FUNCTION "Gest Aut Robot Boxing DX" : VOID
TITLE =Gestione Ciclo Automatico Robot 3 Piantaggi
AUTHOR : MassimoZ
FAMILY : NovaSrl
VERSION : 0.1

BEGIN
NETWORK
TITLE ======== CICLO BOXING DX ======



NETWORK
TITLE ======== Primo Prelievo Ciclo 3 Pinataggi Boxing =======



NETWORK
TITLE =Com Aut Start Primo Posizionamento di Prelievo Asse X Boxing DX
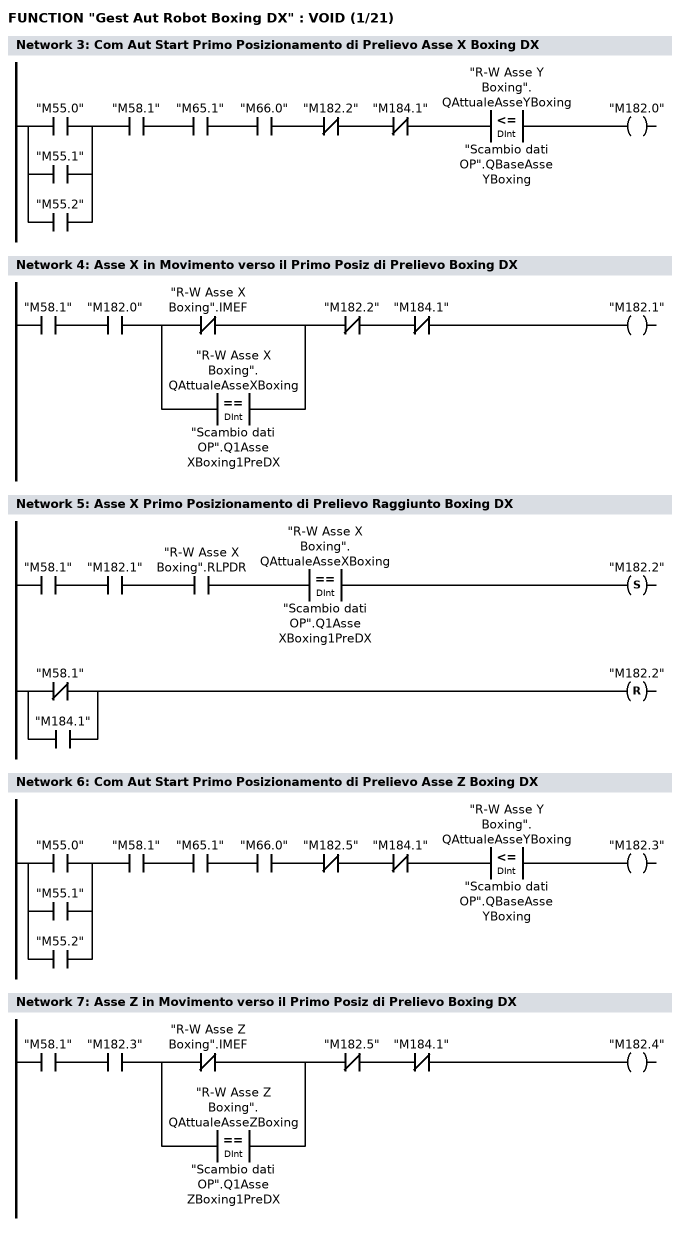
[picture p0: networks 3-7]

      U(    ;
      O     "M55.0";
      O     "M55.1";
      O     "M55.2";
      )     ;
      U     "M58.1";
      U     "M65.1";
      U     "M66.0";
      UN    "M182.2";
      UN    "M184.1";
      U(    ;
      L     "R-W Asse Y Boxing".QAttualeAsseYBoxing;
      L     "Scambio dati OP".QBaseAsseYBoxing;
      <=D   ;
      )     ;
      =     "M182.0";
NETWORK
TITLE =Asse X in Movimento verso il Primo Posiz di Prelievo Boxing DX

      U     "M58.1";
      U     "M182.0";
      U(    ;
      ON    "R-W Asse X Boxing".IMEF;
      O(    ;
      L     "R-W Asse X Boxing".QAttualeAsseXBoxing;
      L     "Scambio dati OP".Q1AsseXBoxing1PreDX;
      ==D   ;
      )     ;
      )     ;
      UN    "M182.2";
      UN    "M184.1";
      =     "M182.1";
NETWORK
TITLE =Asse X Primo Posizionamento di Prelievo Raggiunto Boxing DX

      U     "M58.1";
      U     "M182.1";
      U     "R-W Asse X Boxing".RLPDR;
      U(    ;
      L     "R-W Asse X Boxing".QAttualeAsseXBoxing;
      L     "Scambio dati OP".Q1AsseXBoxing1PreDX;
      ==D   ;
      )     ;
      S     "M182.2";
      U(    ;
      ON    "M58.1";
      O     "M184.1";
      )     ;
      R     "M182.2";
      NOP   0;
NETWORK
TITLE =Com Aut Start Primo Posizionamento di Prelievo Asse Z Boxing DX

      U(    ;
      O     "M55.0";
      O     "M55.1";
      O     "M55.2";
      )     ;
      U     "M58.1";
      U     "M65.1";
      U     "M66.0";
      UN    "M182.5";
      UN    "M184.1";
      U(    ;
      L     "R-W Asse Y Boxing".QAttualeAsseYBoxing;
      L     "Scambio dati OP".QBaseAsseYBoxing;
      <=D   ;
      )     ;
      =     "M182.3";
NETWORK
TITLE =Asse Z in Movimento verso il Primo Posiz di Prelievo Boxing DX

      U     "M58.1";
      U     "M182.3";
      U(    ;
      ON    "R-W Asse Z Boxing".IMEF;
      O(    ;
      L     "R-W Asse Z Boxing".QAttualeAsseZBoxing;
      L     "Scambio dati OP".Q1AsseZBoxing1PreDX;
      ==D   ;
      )     ;
      )     ;
      UN    "M182.5";
      UN    "M184.1";
      =     "M182.4";
NETWORK
TITLE =Asse Z Primo Posizionamento di Prelievo Raggiunto Boxing DX
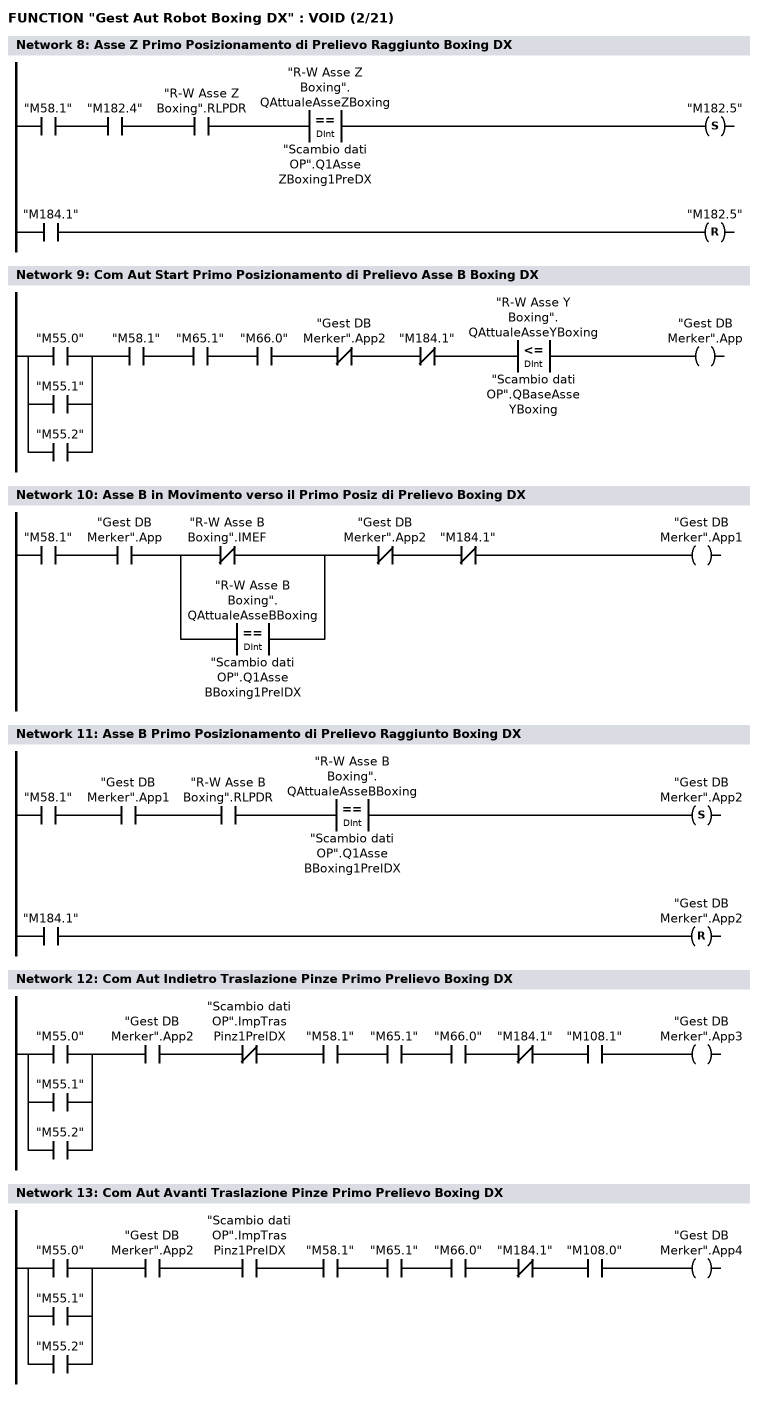
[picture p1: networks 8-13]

      U     "M58.1";
      U     "M182.4";
      U     "R-W Asse Z Boxing".RLPDR;
      U(    ;
      L     "R-W Asse Z Boxing".QAttualeAsseZBoxing;
      L     "Scambio dati OP".Q1AsseZBoxing1PreDX;
      ==D   ;
      )     ;
      S     "M182.5";
      U     "M184.1";
      R     "M182.5";
      NOP   0;
NETWORK
TITLE =Com Aut Start Primo Posizionamento di Prelievo Asse B Boxing DX



      U(    ;
      O     "M55.0";
      O     "M55.1";
      O     "M55.2";
      )     ;
      U     "M58.1";
      U     "M65.1";
      U     "M66.0";
      UN    "Gest DB Merker".App2;
      UN    "M184.1";
      U(    ;
      L     "R-W Asse Y Boxing".QAttualeAsseYBoxing;
      L     "Scambio dati OP".QBaseAsseYBoxing;
      <=D   ;
      )     ;
      =     "Gest DB Merker".App;
NETWORK
TITLE =Asse B in Movimento verso il Primo Posiz di Prelievo Boxing DX

      U     "M58.1";
      U     "Gest DB Merker".App;
      U(    ;
      ON    "R-W Asse B Boxing".IMEF;
      O(    ;
      L     "R-W Asse B Boxing".QAttualeAsseBBoxing;
      L     "Scambio dati OP".Q1AsseBBoxing1PrelDX;
      ==D   ;
      )     ;
      )     ;
      UN    "Gest DB Merker".App2;
      UN    "M184.1";
      =     "Gest DB Merker".App1;
NETWORK
TITLE =Asse B Primo Posizionamento di Prelievo Raggiunto Boxing DX

      U     "M58.1";
      U     "Gest DB Merker".App1;
      U     "R-W Asse B Boxing".RLPDR;
      U(    ;
      L     "R-W Asse B Boxing".QAttualeAsseBBoxing;
      L     "Scambio dati OP".Q1AsseBBoxing1PrelDX;
      ==D   ;
      )     ;
      S     "Gest DB Merker".App2;
      U     "M184.1";
      R     "Gest DB Merker".App2;
      NOP   0;
NETWORK
TITLE =Com Aut Indietro Traslazione Pinze Primo Prelievo Boxing DX

      U(    ;
      O     "M55.0";
      O     "M55.1";
      O     "M55.2";
      )     ;
      U     "Gest DB Merker".App2;
      UN    "Scambio dati OP".ImpTrasPinz1PrelDX;
      U     "M58.1";
      U     "M65.1";
      U     "M66.0";
      UN    "M184.1";
      U     "M108.1";
      =     "Gest DB Merker".App3;
NETWORK
TITLE =Com Aut Avanti Traslazione Pinze Primo Prelievo Boxing DX

      U(    ;
      O     "M55.0";
      O     "M55.1";
      O     "M55.2";
      )     ;
      U     "Gest DB Merker".App2;
      U     "Scambio dati OP".ImpTrasPinz1PrelDX;
      U     "M58.1";
      U     "M65.1";
      U     "M66.0";
      UN    "M184.1";
      U     "M108.0";
      =     "Gest DB Merker".App4;
NETWORK
TITLE =Com Aut Apertura Pinze Primo Prelievo Boxing DX
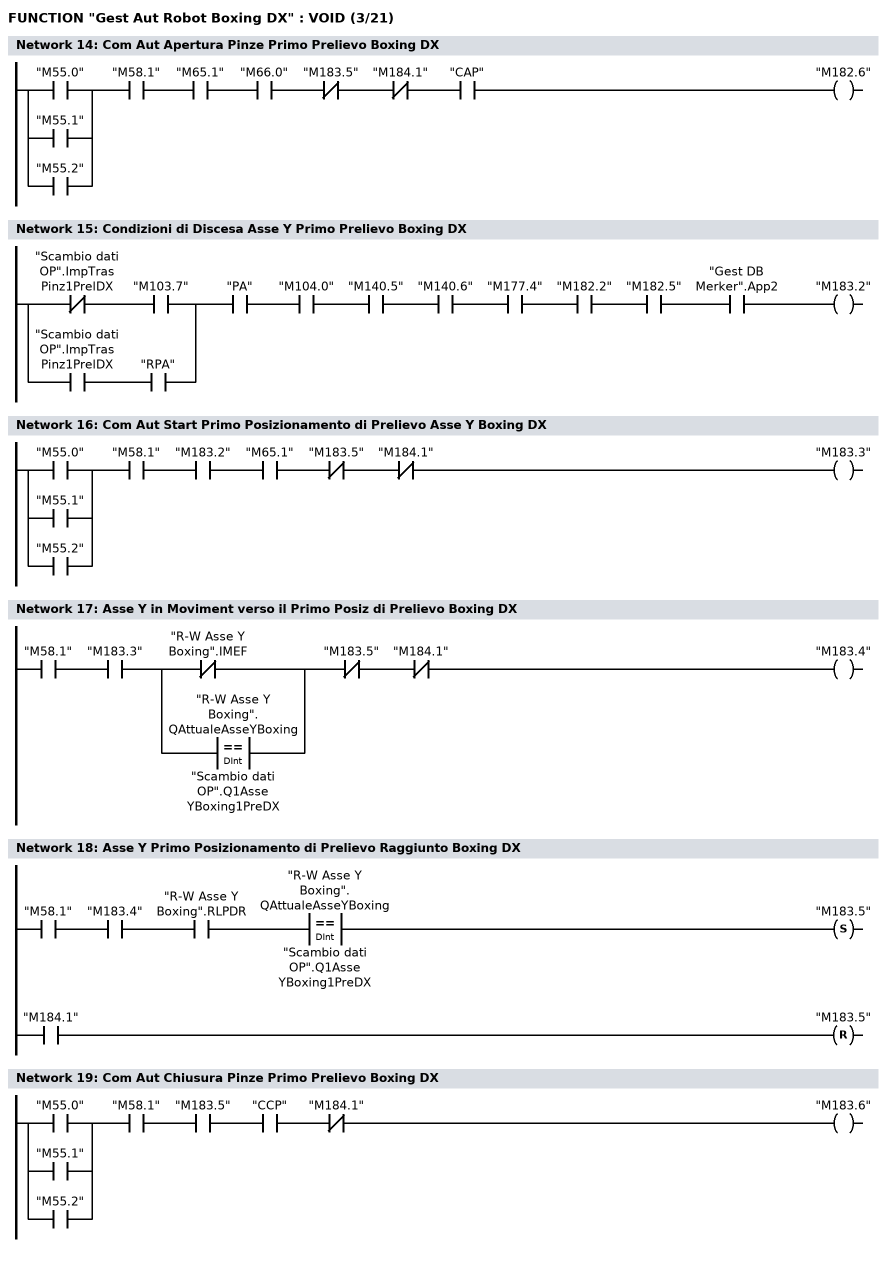
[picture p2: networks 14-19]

      U(    ;
      O     "M55.0";
      O     "M55.1";
      O     "M55.2";
      )     ;
      U     "M58.1";
      U     "M65.1";
      U     "M66.0";
      UN    "M183.5";
      UN    "M184.1";
      U     "CAP";
      =     "M182.6";
NETWORK
TITLE =Condizioni di Discesa Asse Y Primo Prelievo Boxing DX

      U(    ;
      UN    "Scambio dati OP".ImpTrasPinz1PrelDX;
      U     "M103.7";
      O     ;
      U     "Scambio dati OP".ImpTrasPinz1PrelDX;
      U     "RPA";
      )     ;
      U     "PA";
      U     "M104.0";
      U     "M140.5";
      U     "M140.6";
      U     "M177.4";
      U     "M182.2";
      U     "M182.5";
      U     "Gest DB Merker".App2;
      =     "M183.2";
NETWORK
TITLE =Com Aut Start Primo Posizionamento di Prelievo Asse Y Boxing DX

      U(    ;
      O     "M55.0";
      O     "M55.1";
      O     "M55.2";
      )     ;
      U     "M58.1";
      U     "M183.2";
      U     "M65.1";
      UN    "M183.5";
      UN    "M184.1";
      =     "M183.3";
NETWORK
TITLE =Asse Y in Moviment verso il Primo Posiz di Prelievo Boxing DX

      U     "M58.1";
      U     "M183.3";
      U(    ;
      ON    "R-W Asse Y Boxing".IMEF;
      O(    ;
      L     "R-W Asse Y Boxing".QAttualeAsseYBoxing;
      L     "Scambio dati OP".Q1AsseYBoxing1PreDX;
      ==D   ;
      )     ;
      )     ;
      UN    "M183.5";
      UN    "M184.1";
      =     "M183.4";
NETWORK
TITLE =Asse Y Primo Posizionamento di Prelievo Raggiunto Boxing DX

      U     "M58.1";
      U     "M183.4";
      U     "R-W Asse Y Boxing".RLPDR;
      U(    ;
      L     "R-W Asse Y Boxing".QAttualeAsseYBoxing;
      L     "Scambio dati OP".Q1AsseYBoxing1PreDX;
      ==D   ;
      )     ;
      S     "M183.5";
      U     "M184.1";
      R     "M183.5";
      NOP   0;
NETWORK
TITLE =Com Aut Chiusura Pinze Primo Prelievo Boxing DX

      U(    ;
      O     "M55.0";
      O     "M55.1";
      O     "M55.2";
      )     ;
      U     "M58.1";
      U     "M183.5";
      U     "CCP";
      UN    "M184.1";
      =     "M183.6";
NETWORK
TITLE =Tempo Chiusura Pinze Primo Prelievo Boxing DX
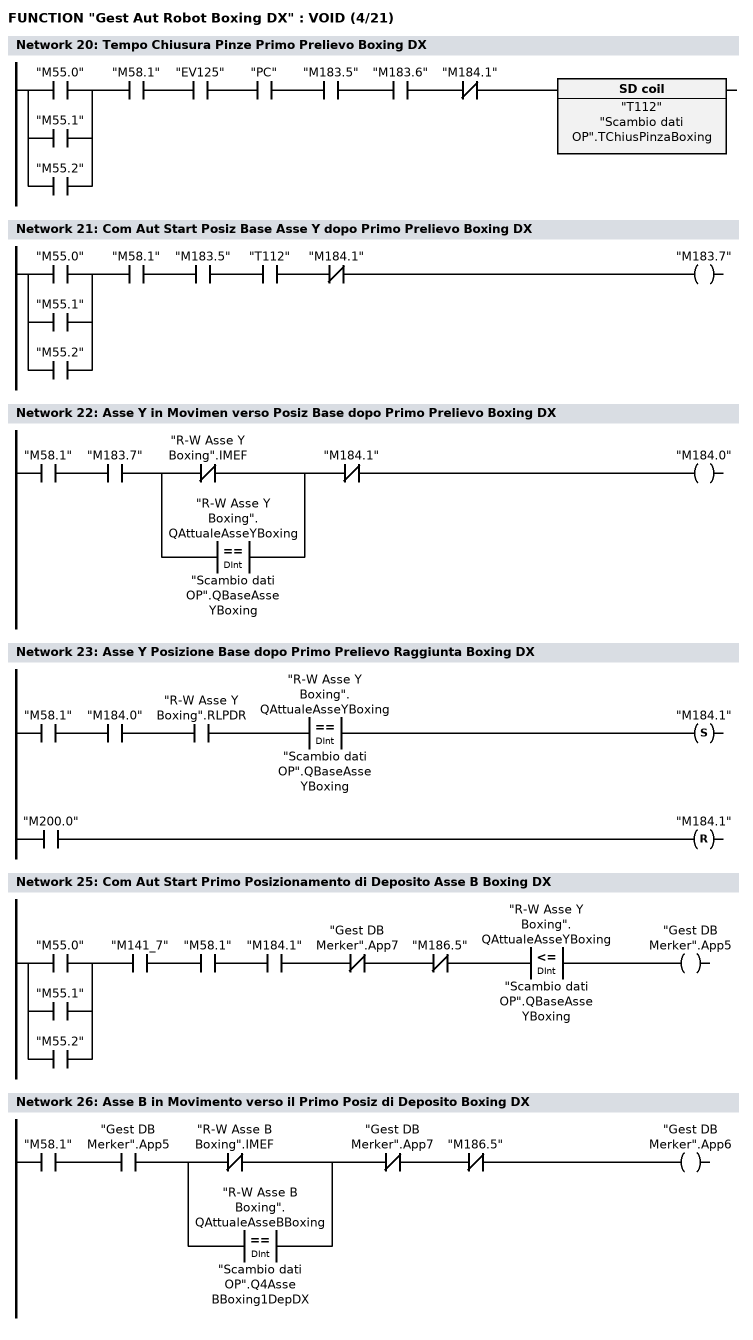
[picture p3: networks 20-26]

      U(    ;
      O     "M55.0";
      O     "M55.1";
      O     "M55.2";
      )     ;
      U     "M58.1";
      U     "EV125";
      U     "PC";
      U     "M183.5";
      U     "M183.6";
      UN    "M184.1";
      L     "Scambio dati OP".TChiusPinzaBoxing;
      SE    "T112";
      NOP   0;
      NOP   0;
      NOP   0;
      NOP   0;
NETWORK
TITLE =Com Aut Start Posiz Base Asse Y dopo Primo Prelievo Boxing DX

      U(    ;
      O     "M55.0";
      O     "M55.1";
      O     "M55.2";
      )     ;
      U     "M58.1";
      U     "M183.5";
      U     "T112";
      UN    "M184.1";
      =     "M183.7";
NETWORK
TITLE =Asse Y in Movimen verso Posiz Base dopo Primo Prelievo Boxing DX

      U     "M58.1";
      U     "M183.7";
      U(    ;
      ON    "R-W Asse Y Boxing".IMEF;
      O(    ;
      L     "R-W Asse Y Boxing".QAttualeAsseYBoxing;
      L     "Scambio dati OP".QBaseAsseYBoxing;
      ==D   ;
      )     ;
      )     ;
      UN    "M184.1";
      =     "M184.0";
NETWORK
TITLE =Asse Y Posizione Base dopo Primo Prelievo Raggiunta Boxing DX

      U     "M58.1";
      U     "M184.0";
      U     "R-W Asse Y Boxing".RLPDR;
      U(    ;
      L     "R-W Asse Y Boxing".QAttualeAsseYBoxing;
      L     "Scambio dati OP".QBaseAsseYBoxing;
      ==D   ;
      )     ;
      S     "M184.1";
      U     "M200.0";
      R     "M184.1";
      NOP   0;
NETWORK
TITLE ======== Primo Deposito Ciclo 3 Pinataggi Boxing =======



NETWORK
TITLE =Com Aut Start Primo Posizionamento di Deposito Asse B Boxing DX

      U(    ;
      O     "M55.0";
      O     "M55.1";
      O     "M55.2";
      )     ;
      U     "M141_7";
      U     "M58.1";
      U     "M184.1";
      UN    "Gest DB Merker".App7;
      UN    "M186.5";
      U(    ;
      L     "R-W Asse Y Boxing".QAttualeAsseYBoxing;
      L     "Scambio dati OP".QBaseAsseYBoxing;
      <=D   ;
      )     ;
      =     "Gest DB Merker".App5;
NETWORK
TITLE =Asse B in Movimento verso il Primo Posiz di Deposito Boxing DX

      U     "M58.1";
      U     "Gest DB Merker".App5;
      U(    ;
      ON    "R-W Asse B Boxing".IMEF;
      O(    ;
      L     "R-W Asse B Boxing".QAttualeAsseBBoxing;
      L     "Scambio dati OP".Q4AsseBBoxing1DepDX;
      ==D   ;
      )     ;
      )     ;
      UN    "Gest DB Merker".App7;
      UN    "M186.5";
      =     "Gest DB Merker".App6;
NETWORK
TITLE =Asse B Primo Posizionamento di Deposito Raggiunto Boxing DX
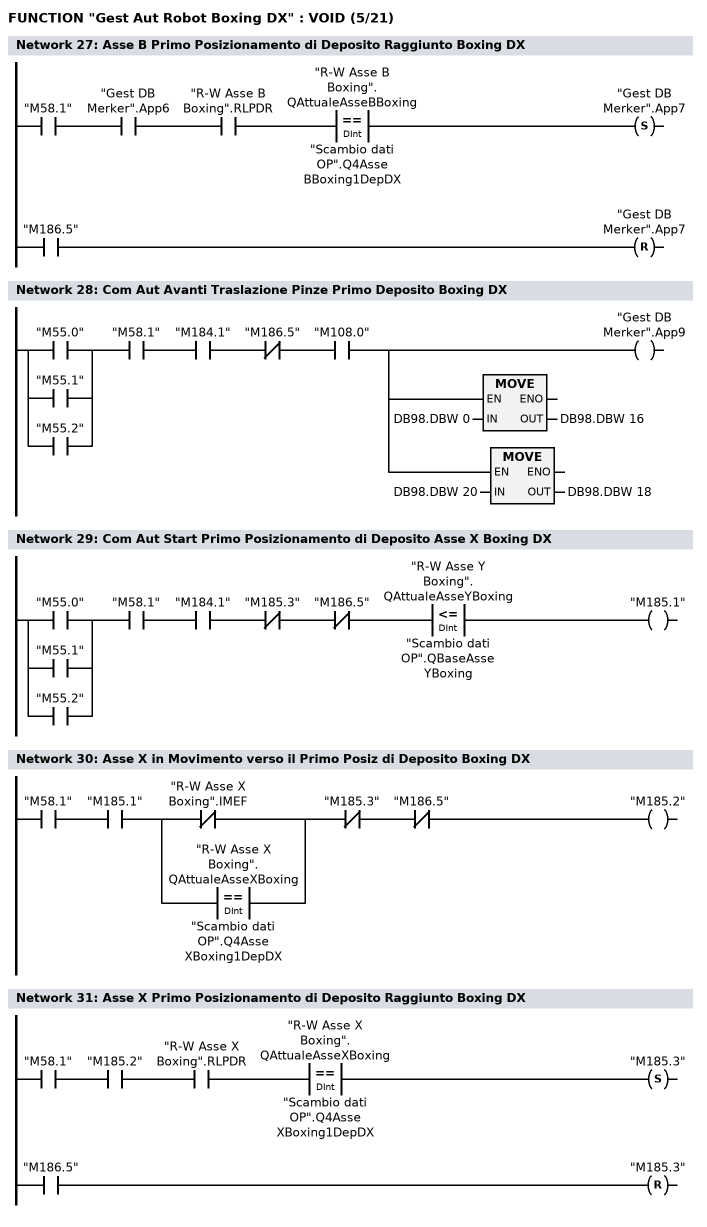
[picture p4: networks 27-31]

      U     "M58.1";
      U     "Gest DB Merker".App6;
      U     "R-W Asse B Boxing".RLPDR;
      U(    ;
      L     "R-W Asse B Boxing".QAttualeAsseBBoxing;
      L     "Scambio dati OP".Q4AsseBBoxing1DepDX;
      ==D   ;
      )     ;
      S     "Gest DB Merker".App7;
      U     "M186.5";
      R     "Gest DB Merker".App7;
      NOP   0;
NETWORK
TITLE =Com Aut Avanti Traslazione Pinze Primo Deposito Boxing DX

      U(    ;
      O     "M55.0";
      O     "M55.1";
      O     "M55.2";
      )     ;
      U     "M58.1";
      U     "M184.1";
      UN    "M186.5";
      U     "M108.0";
      =     L      0.0;
      U     L      0.0;
      BLD   102;
      =     "Gest DB Merker".App9;
      U     L      0.0;
      SPBNB _001;
      L     DB98.DBW    0;
      T     DB98.DBW   16;
_001: NOP   0;
      U     L      0.0;
      SPBNB _002;
      L     DB98.DBW   20;
      T     DB98.DBW   18;
_002: NOP   0;
NETWORK
TITLE =Com Aut Start Primo Posizionamento di Deposito Asse X Boxing DX

      U(    ;
      O     "M55.0";
      O     "M55.1";
      O     "M55.2";
      )     ;
      U     "M58.1";
      U     "M184.1";
      UN    "M185.3";
      UN    "M186.5";
      U(    ;
      L     "R-W Asse Y Boxing".QAttualeAsseYBoxing;
      L     "Scambio dati OP".QBaseAsseYBoxing;
      <=D   ;
      )     ;
      =     "M185.1";
NETWORK
TITLE =Asse X in Movimento verso il Primo Posiz di Deposito Boxing DX

      U     "M58.1";
      U     "M185.1";
      U(    ;
      ON    "R-W Asse X Boxing".IMEF;
      O(    ;
      L     "R-W Asse X Boxing".QAttualeAsseXBoxing;
      L     "Scambio dati OP".Q4AsseXBoxing1DepDX;
      ==D   ;
      )     ;
      )     ;
      UN    "M185.3";
      UN    "M186.5";
      =     "M185.2";
NETWORK
TITLE =Asse X Primo Posizionamento di Deposito Raggiunto Boxing DX

      U     "M58.1";
      U     "M185.2";
      U     "R-W Asse X Boxing".RLPDR;
      U(    ;
      L     "R-W Asse X Boxing".QAttualeAsseXBoxing;
      L     "Scambio dati OP".Q4AsseXBoxing1DepDX;
      ==D   ;
      )     ;
      S     "M185.3";
      U     "M186.5";
      R     "M185.3";
      NOP   0;
NETWORK
TITLE =Com Aut Start Primo Posizionamento di Deposito Asse Z Boxing DX
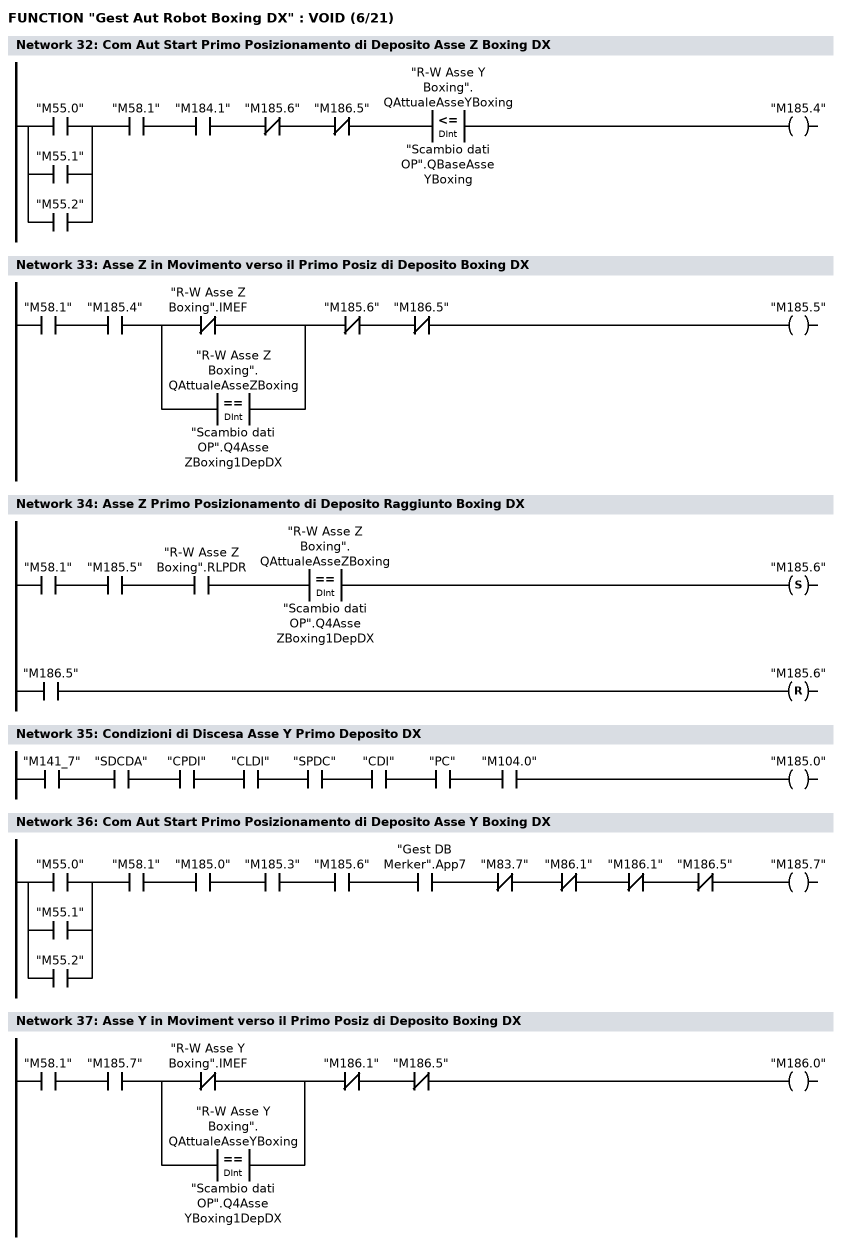
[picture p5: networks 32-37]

      U(    ;
      O     "M55.0";
      O     "M55.1";
      O     "M55.2";
      )     ;
      U     "M58.1";
      U     "M184.1";
      UN    "M185.6";
      UN    "M186.5";
      U(    ;
      L     "R-W Asse Y Boxing".QAttualeAsseYBoxing;
      L     "Scambio dati OP".QBaseAsseYBoxing;
      <=D   ;
      )     ;
      =     "M185.4";
NETWORK
TITLE =Asse Z in Movimento verso il Primo Posiz di Deposito Boxing DX

      U     "M58.1";
      U     "M185.4";
      U(    ;
      ON    "R-W Asse Z Boxing".IMEF;
      O(    ;
      L     "R-W Asse Z Boxing".QAttualeAsseZBoxing;
      L     "Scambio dati OP".Q4AsseZBoxing1DepDX;
      ==D   ;
      )     ;
      )     ;
      UN    "M185.6";
      UN    "M186.5";
      =     "M185.5";
NETWORK
TITLE =Asse Z Primo Posizionamento di Deposito Raggiunto Boxing DX

      U     "M58.1";
      U     "M185.5";
      U     "R-W Asse Z Boxing".RLPDR;
      U(    ;
      L     "R-W Asse Z Boxing".QAttualeAsseZBoxing;
      L     "Scambio dati OP".Q4AsseZBoxing1DepDX;
      ==D   ;
      )     ;
      S     "M185.6";
      U     "M186.5";
      R     "M185.6";
      NOP   0;
NETWORK
TITLE =Condizioni di Discesa Asse Y Primo Deposito DX

      U     "M141_7";
      U     "SDCDA";
      U     "CPDI";
      U     "CLDI";
      U     "SPDC";
      U     "CDI";
      U     "PC";
      U     "M104.0";
      =     "M185.0";
NETWORK
TITLE =Com Aut Start Primo Posizionamento di Deposito Asse Y Boxing DX

      U(    ;
      O     "M55.0";
      O     "M55.1";
      O     "M55.2";
      )     ;
      U     "M58.1";
      U     "M185.0";
      U     "M185.3";
      U     "M185.6";
      U     "Gest DB Merker".App7;
      UN    "M83.7";
      UN    "M86.1";
      UN    "M186.1";
      UN    "M186.5";
      =     "M185.7";
NETWORK
TITLE =Asse Y in Moviment verso il Primo Posiz di Deposito Boxing DX

      U     "M58.1";
      U     "M185.7";
      U(    ;
      ON    "R-W Asse Y Boxing".IMEF;
      O(    ;
      L     "R-W Asse Y Boxing".QAttualeAsseYBoxing;
      L     "Scambio dati OP".Q4AsseYBoxing1DepDX;
      ==D   ;
      )     ;
      )     ;
      UN    "M186.1";
      UN    "M186.5";
      =     "M186.0";
NETWORK
TITLE =Asse Y Primo Posizionamento di Deposito Raggiunto Boxing DX
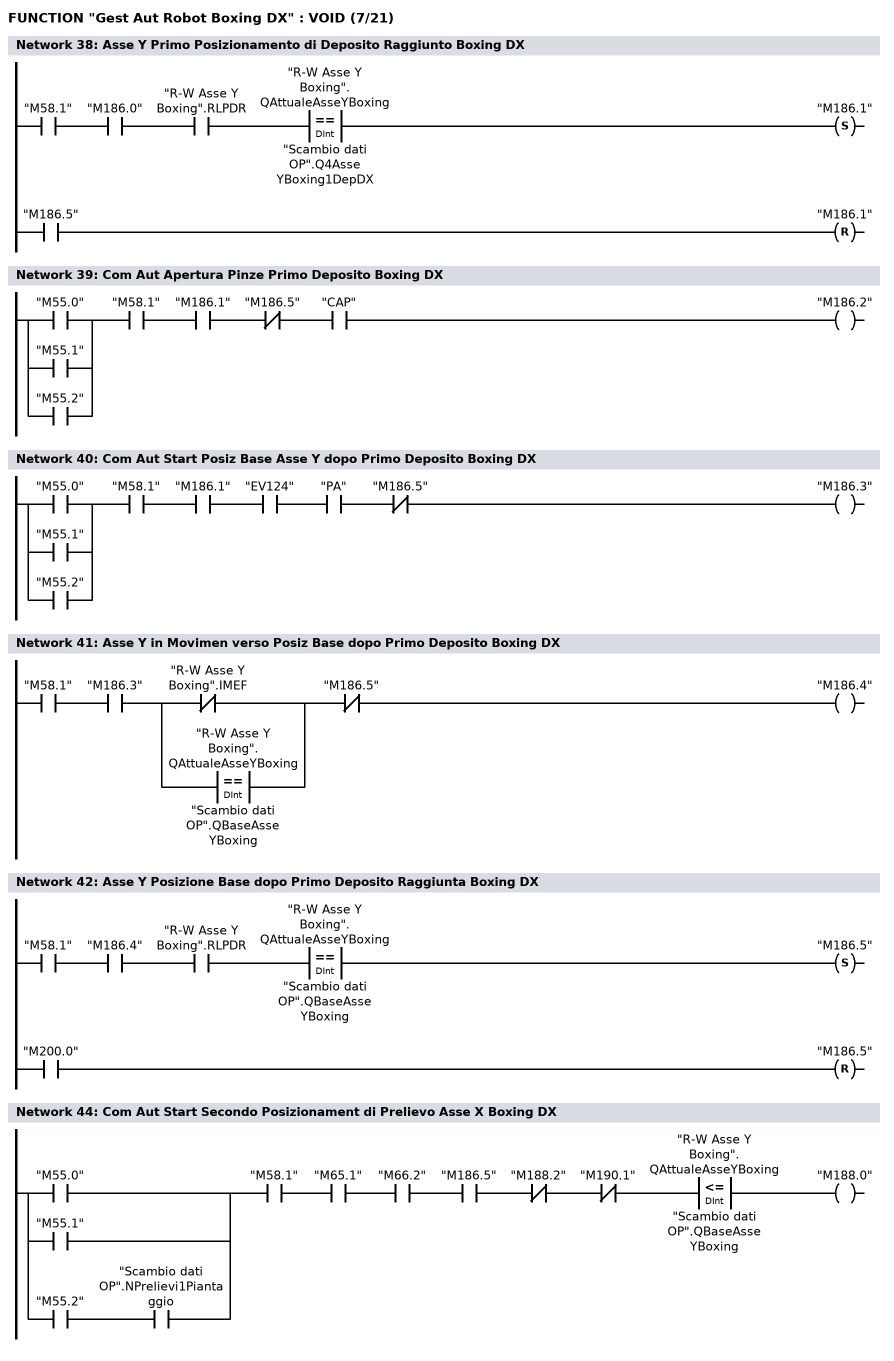
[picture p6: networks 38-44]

      U     "M58.1";
      U     "M186.0";
      U     "R-W Asse Y Boxing".RLPDR;
      U(    ;
      L     "R-W Asse Y Boxing".QAttualeAsseYBoxing;
      L     "Scambio dati OP".Q4AsseYBoxing1DepDX;
      ==D   ;
      )     ;
      S     "M186.1";
      U     "M186.5";
      R     "M186.1";
      NOP   0;
NETWORK
TITLE =Com Aut Apertura Pinze Primo Deposito Boxing DX

      U(    ;
      O     "M55.0";
      O     "M55.1";
      O     "M55.2";
      )     ;
      U     "M58.1";
      U     "M186.1";
      UN    "M186.5";
      U     "CAP";
      =     "M186.2";
NETWORK
TITLE =Com Aut Start Posiz Base Asse Y dopo Primo Deposito Boxing DX

      U(    ;
      O     "M55.0";
      O     "M55.1";
      O     "M55.2";
      )     ;
      U     "M58.1";
      U     "M186.1";
      U     "EV124";
      U     "PA";
      UN    "M186.5";
      =     "M186.3";
NETWORK
TITLE =Asse Y in Movimen verso Posiz Base dopo Primo Deposito Boxing DX

      U     "M58.1";
      U     "M186.3";
      U(    ;
      ON    "R-W Asse Y Boxing".IMEF;
      O(    ;
      L     "R-W Asse Y Boxing".QAttualeAsseYBoxing;
      L     "Scambio dati OP".QBaseAsseYBoxing;
      ==D   ;
      )     ;
      )     ;
      UN    "M186.5";
      =     "M186.4";
NETWORK
TITLE =Asse Y Posizione Base dopo Primo Deposito Raggiunta Boxing DX

      U     "M58.1";
      U     "M186.4";
      U     "R-W Asse Y Boxing".RLPDR;
      U(    ;
      L     "R-W Asse Y Boxing".QAttualeAsseYBoxing;
      L     "Scambio dati OP".QBaseAsseYBoxing;
      ==D   ;
      )     ;
      S     "M186.5";
      U     "M200.0";
      R     "M186.5";
      NOP   0;
NETWORK
TITLE ======== Secondo Prelievo Ciclo 3 Pinataggi Boxing =======



NETWORK
TITLE =Com Aut Start Secondo Posizionament di Prelievo Asse X Boxing DX

      U(    ;
      O     "M55.0";
      O     "M55.1";
      O     ;
      U     "M55.2";
      U     "Scambio dati OP".NPrelievi1Piantaggio;
      )     ;
      U     "M58.1";
      U     "M65.1";
      U     "M66.2";
      U     "M186.5";
      UN    "M188.2";
      UN    "M190.1";
      U(    ;
      L     "R-W Asse Y Boxing".QAttualeAsseYBoxing;
      L     "Scambio dati OP".QBaseAsseYBoxing;
      <=D   ;
      )     ;
      =     "M188.0";
NETWORK
TITLE =Asse X in Movimento verso il Secondo Posiz di Prelievo Boxing DX
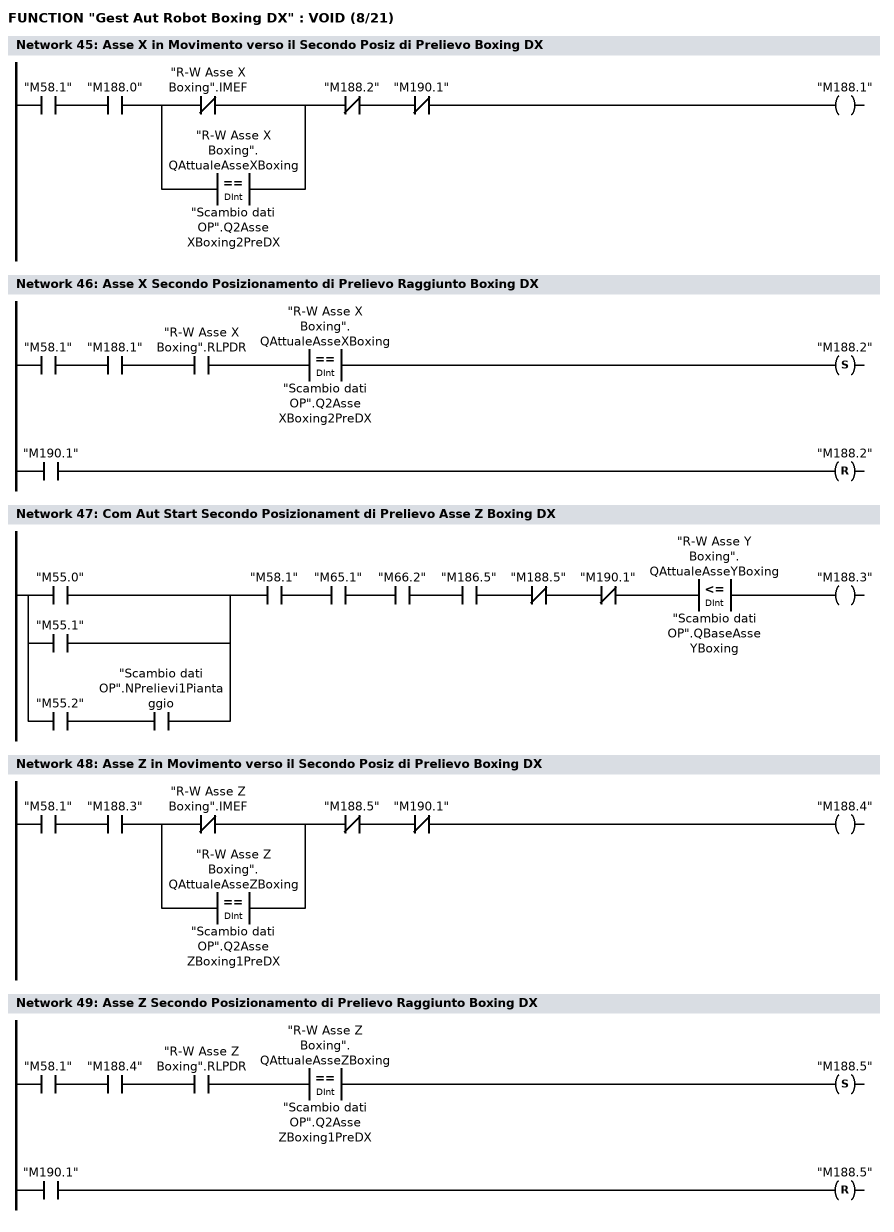
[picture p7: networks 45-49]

      U     "M58.1";
      U     "M188.0";
      U(    ;
      ON    "R-W Asse X Boxing".IMEF;
      O(    ;
      L     "R-W Asse X Boxing".QAttualeAsseXBoxing;
      L     "Scambio dati OP".Q2AsseXBoxing2PreDX;
      ==D   ;
      )     ;
      )     ;
      UN    "M188.2";
      UN    "M190.1";
      =     "M188.1";
NETWORK
TITLE =Asse X Secondo Posizionamento di Prelievo Raggiunto Boxing DX

      U     "M58.1";
      U     "M188.1";
      U     "R-W Asse X Boxing".RLPDR;
      U(    ;
      L     "R-W Asse X Boxing".QAttualeAsseXBoxing;
      L     "Scambio dati OP".Q2AsseXBoxing2PreDX;
      ==D   ;
      )     ;
      S     "M188.2";
      U     "M190.1";
      R     "M188.2";
      NOP   0;
NETWORK
TITLE =Com Aut Start Secondo Posizionament di Prelievo Asse Z Boxing DX

      U(    ;
      O     "M55.0";
      O     "M55.1";
      O     ;
      U     "M55.2";
      U     "Scambio dati OP".NPrelievi1Piantaggio;
      )     ;
      U     "M58.1";
      U     "M65.1";
      U     "M66.2";
      U     "M186.5";
      UN    "M188.5";
      UN    "M190.1";
      U(    ;
      L     "R-W Asse Y Boxing".QAttualeAsseYBoxing;
      L     "Scambio dati OP".QBaseAsseYBoxing;
      <=D   ;
      )     ;
      =     "M188.3";
NETWORK
TITLE =Asse Z in Movimento verso il Secondo Posiz di Prelievo Boxing DX

      U     "M58.1";
      U     "M188.3";
      U(    ;
      ON    "R-W Asse Z Boxing".IMEF;
      O(    ;
      L     "R-W Asse Z Boxing".QAttualeAsseZBoxing;
      L     "Scambio dati OP".Q2AsseZBoxing1PreDX;
      ==D   ;
      )     ;
      )     ;
      UN    "M188.5";
      UN    "M190.1";
      =     "M188.4";
NETWORK
TITLE =Asse Z Secondo Posizionamento di Prelievo Raggiunto Boxing DX

      U     "M58.1";
      U     "M188.4";
      U     "R-W Asse Z Boxing".RLPDR;
      U(    ;
      L     "R-W Asse Z Boxing".QAttualeAsseZBoxing;
      L     "Scambio dati OP".Q2AsseZBoxing1PreDX;
      ==D   ;
      )     ;
      S     "M188.5";
      U     "M190.1";
      R     "M188.5";
      NOP   0;
NETWORK
TITLE =Com Aut Start Secondo Posizionament di Prelievo Asse B Boxing DX
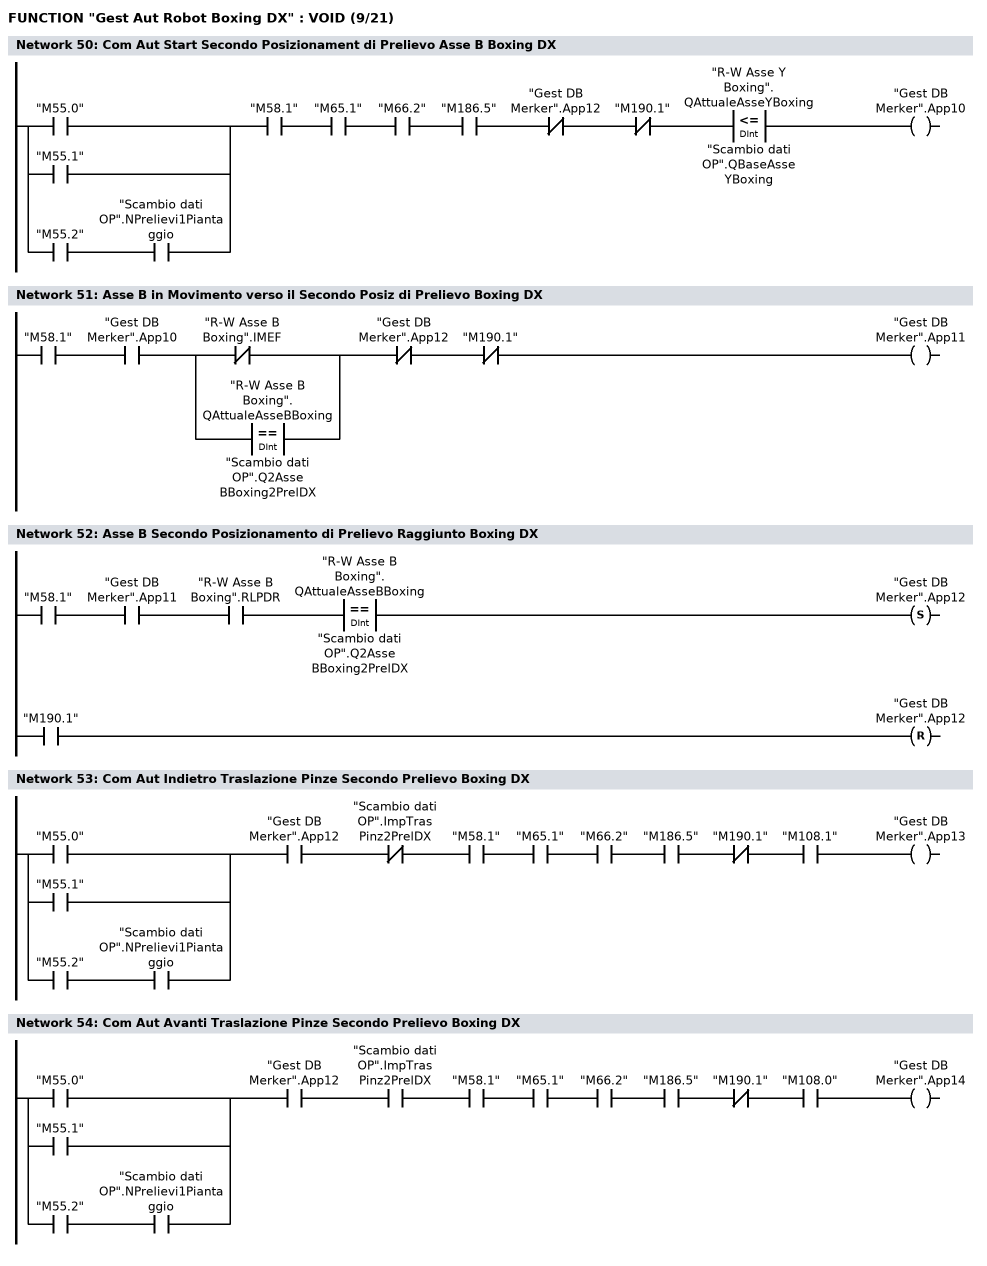
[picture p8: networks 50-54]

      U(    ;
      O     "M55.0";
      O     "M55.1";
      O     ;
      U     "M55.2";
      U     "Scambio dati OP".NPrelievi1Piantaggio;
      )     ;
      U     "M58.1";
      U     "M65.1";
      U     "M66.2";
      U     "M186.5";
      UN    "Gest DB Merker".App12;
      UN    "M190.1";
      U(    ;
      L     "R-W Asse Y Boxing".QAttualeAsseYBoxing;
      L     "Scambio dati OP".QBaseAsseYBoxing;
      <=D   ;
      )     ;
      =     "Gest DB Merker".App10;
NETWORK
TITLE =Asse B in Movimento verso il Secondo Posiz di Prelievo Boxing DX

      U     "M58.1";
      U     "Gest DB Merker".App10;
      U(    ;
      ON    "R-W Asse B Boxing".IMEF;
      O(    ;
      L     "R-W Asse B Boxing".QAttualeAsseBBoxing;
      L     "Scambio dati OP".Q2AsseBBoxing2PrelDX;
      ==D   ;
      )     ;
      )     ;
      UN    "Gest DB Merker".App12;
      UN    "M190.1";
      =     "Gest DB Merker".App11;
NETWORK
TITLE =Asse B Secondo Posizionamento di Prelievo Raggiunto Boxing DX

      U     "M58.1";
      U     "Gest DB Merker".App11;
      U     "R-W Asse B Boxing".RLPDR;
      U(    ;
      L     "R-W Asse B Boxing".QAttualeAsseBBoxing;
      L     "Scambio dati OP".Q2AsseBBoxing2PrelDX;
      ==D   ;
      )     ;
      S     "Gest DB Merker".App12;
      U     "M190.1";
      R     "Gest DB Merker".App12;
      NOP   0;
NETWORK
TITLE =Com Aut Indietro Traslazione Pinze Secondo Prelievo Boxing DX

      U(    ;
      O     "M55.0";
      O     "M55.1";
      O     ;
      U     "M55.2";
      U     "Scambio dati OP".NPrelievi1Piantaggio;
      )     ;
      U     "Gest DB Merker".App12;
      UN    "Scambio dati OP".ImpTrasPinz2PrelDX;
      U     "M58.1";
      U     "M65.1";
      U     "M66.2";
      U     "M186.5";
      UN    "M190.1";
      U     "M108.1";
      =     "Gest DB Merker".App13;
NETWORK
TITLE =Com Aut Avanti Traslazione Pinze Secondo Prelievo Boxing DX

      U(    ;
      O     "M55.0";
      O     "M55.1";
      O     ;
      U     "M55.2";
      U     "Scambio dati OP".NPrelievi1Piantaggio;
      )     ;
      U     "Gest DB Merker".App12;
      U     "Scambio dati OP".ImpTrasPinz2PrelDX;
      U     "M58.1";
      U     "M65.1";
      U     "M66.2";
      U     "M186.5";
      UN    "M190.1";
      U     "M108.0";
      =     "Gest DB Merker".App14;
NETWORK
TITLE =Com Aut Apertura Pinze Secondo Prelievo Boxing DX
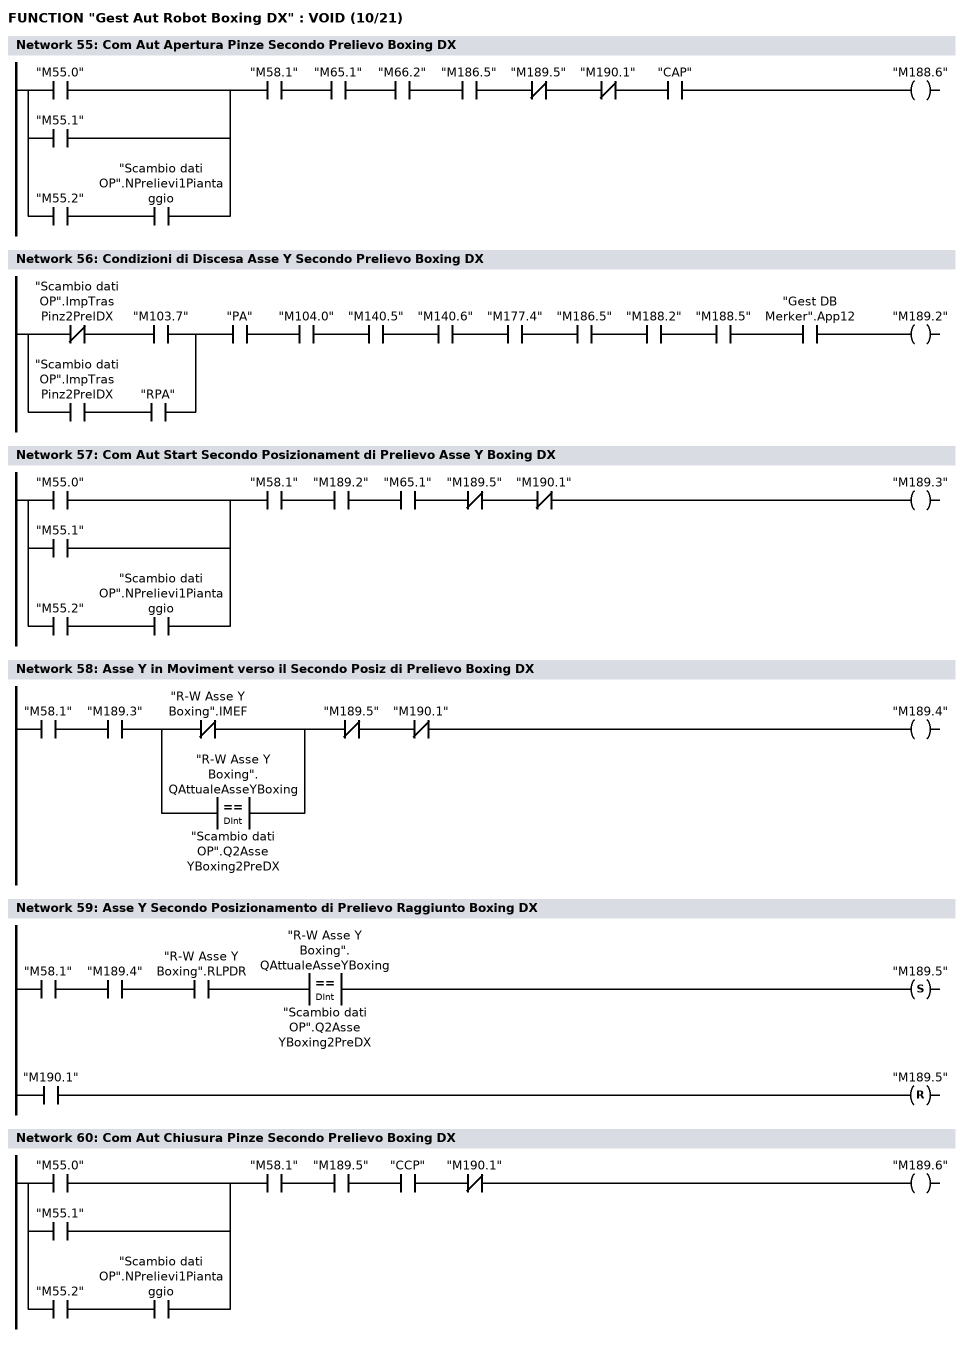
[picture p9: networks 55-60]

      U(    ;
      O     "M55.0";
      O     "M55.1";
      O     ;
      U     "M55.2";
      U     "Scambio dati OP".NPrelievi1Piantaggio;
      )     ;
      U     "M58.1";
      U     "M65.1";
      U     "M66.2";
      U     "M186.5";
      UN    "M189.5";
      UN    "M190.1";
      U     "CAP";
      =     "M188.6";
NETWORK
TITLE =Condizioni di Discesa Asse Y Secondo Prelievo Boxing DX

      U(    ;
      UN    "Scambio dati OP".ImpTrasPinz2PrelDX;
      U     "M103.7";
      O     ;
      U     "Scambio dati OP".ImpTrasPinz2PrelDX;
      U     "RPA";
      )     ;
      U     "PA";
      U     "M104.0";
      U     "M140.5";
      U     "M140.6";
      U     "M177.4";
      U     "M186.5";
      U     "M188.2";
      U     "M188.5";
      U     "Gest DB Merker".App12;
      =     "M189.2";
NETWORK
TITLE =Com Aut Start Secondo Posizionament di Prelievo Asse Y Boxing DX

      U(    ;
      O     "M55.0";
      O     "M55.1";
      O     ;
      U     "M55.2";
      U     "Scambio dati OP".NPrelievi1Piantaggio;
      )     ;
      U     "M58.1";
      U     "M189.2";
      U     "M65.1";
      UN    "M189.5";
      UN    "M190.1";
      =     "M189.3";
NETWORK
TITLE =Asse Y in Moviment verso il Secondo Posiz di Prelievo Boxing DX

      U     "M58.1";
      U     "M189.3";
      U(    ;
      ON    "R-W Asse Y Boxing".IMEF;
      O(    ;
      L     "R-W Asse Y Boxing".QAttualeAsseYBoxing;
      L     "Scambio dati OP".Q2AsseYBoxing2PreDX;
      ==D   ;
      )     ;
      )     ;
      UN    "M189.5";
      UN    "M190.1";
      =     "M189.4";
NETWORK
TITLE =Asse Y Secondo Posizionamento di Prelievo Raggiunto Boxing DX

      U     "M58.1";
      U     "M189.4";
      U     "R-W Asse Y Boxing".RLPDR;
      U(    ;
      L     "R-W Asse Y Boxing".QAttualeAsseYBoxing;
      L     "Scambio dati OP".Q2AsseYBoxing2PreDX;
      ==D   ;
      )     ;
      S     "M189.5";
      U     "M190.1";
      R     "M189.5";
      NOP   0;
NETWORK
TITLE =Com Aut Chiusura Pinze Secondo Prelievo Boxing DX

      U(    ;
      O     "M55.0";
      O     "M55.1";
      O     ;
      U     "M55.2";
      U     "Scambio dati OP".NPrelievi1Piantaggio;
      )     ;
      U     "M58.1";
      U     "M189.5";
      U     "CCP";
      UN    "M190.1";
      =     "M189.6";
NETWORK
TITLE =Tempo Chiusura Pinze Secondo Prelievo Boxing DX
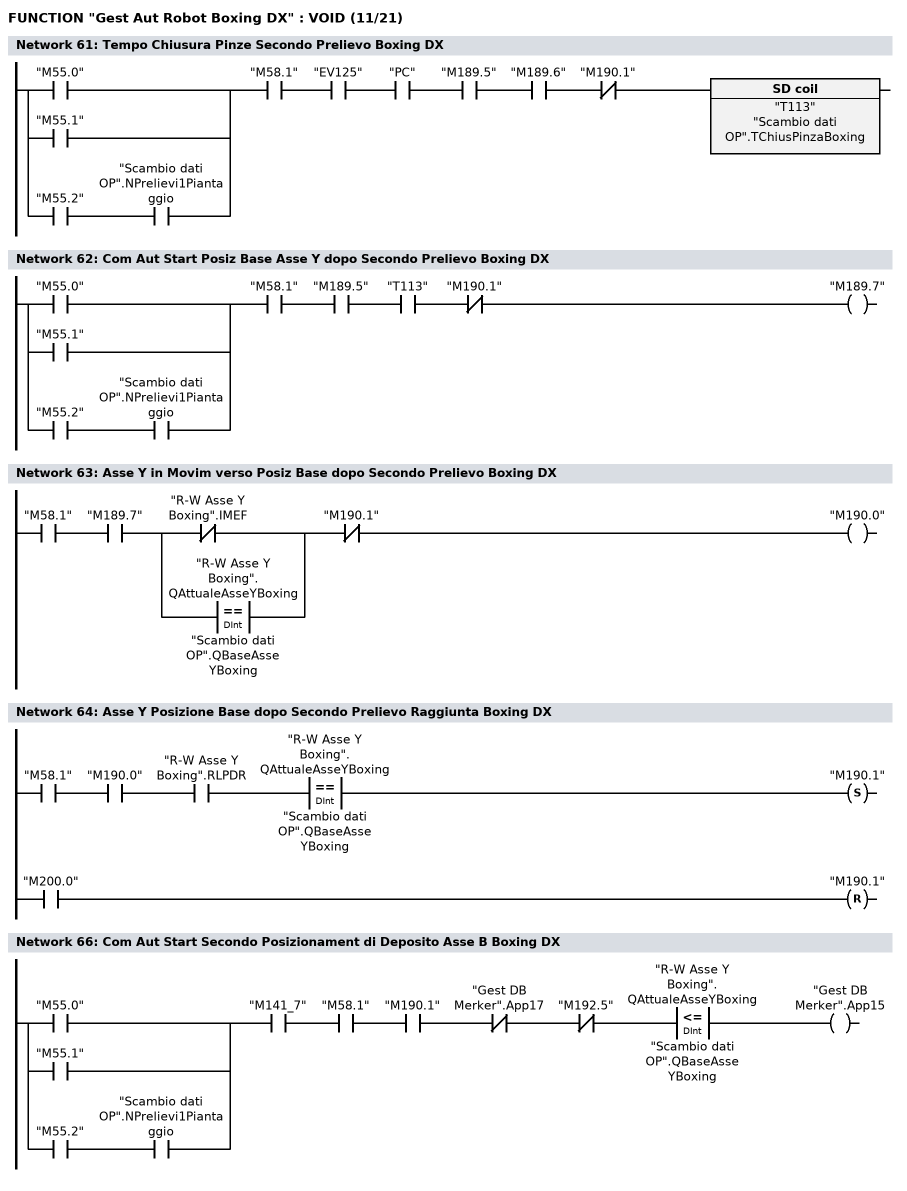
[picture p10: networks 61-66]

      U(    ;
      O     "M55.0";
      O     "M55.1";
      O     ;
      U     "M55.2";
      U     "Scambio dati OP".NPrelievi1Piantaggio;
      )     ;
      U     "M58.1";
      U     "EV125";
      U     "PC";
      U     "M189.5";
      U     "M189.6";
      UN    "M190.1";
      L     "Scambio dati OP".TChiusPinzaBoxing;
      SE    "T113";
      NOP   0;
      NOP   0;
      NOP   0;
      NOP   0;
NETWORK
TITLE =Com Aut Start Posiz Base Asse Y dopo Secondo Prelievo Boxing DX

      U(    ;
      O     "M55.0";
      O     "M55.1";
      O     ;
      U     "M55.2";
      U     "Scambio dati OP".NPrelievi1Piantaggio;
      )     ;
      U     "M58.1";
      U     "M189.5";
      U     "T113";
      UN    "M190.1";
      =     "M189.7";
NETWORK
TITLE =Asse Y in Movim verso Posiz Base dopo Secondo Prelievo Boxing DX

      U     "M58.1";
      U     "M189.7";
      U(    ;
      ON    "R-W Asse Y Boxing".IMEF;
      O(    ;
      L     "R-W Asse Y Boxing".QAttualeAsseYBoxing;
      L     "Scambio dati OP".QBaseAsseYBoxing;
      ==D   ;
      )     ;
      )     ;
      UN    "M190.1";
      =     "M190.0";
NETWORK
TITLE =Asse Y Posizione Base dopo Secondo Prelievo Raggiunta Boxing DX

      U     "M58.1";
      U     "M190.0";
      U     "R-W Asse Y Boxing".RLPDR;
      U(    ;
      L     "R-W Asse Y Boxing".QAttualeAsseYBoxing;
      L     "Scambio dati OP".QBaseAsseYBoxing;
      ==D   ;
      )     ;
      S     "M190.1";
      U     "M200.0";
      R     "M190.1";
      NOP   0;
NETWORK
TITLE ======== Secondo Deposito Ciclo 3 Pinataggi Boxing =======



NETWORK
TITLE =Com Aut Start Secondo Posizionament di Deposito Asse B Boxing DX

      U(    ;
      O     "M55.0";
      O     "M55.1";
      O     ;
      U     "M55.2";
      U     "Scambio dati OP".NPrelievi1Piantaggio;
      )     ;
      U     "M141_7";
      U     "M58.1";
      U     "M190.1";
      UN    "Gest DB Merker".App17;
      UN    "M192.5";
      U(    ;
      L     "R-W Asse Y Boxing".QAttualeAsseYBoxing;
      L     "Scambio dati OP".QBaseAsseYBoxing;
      <=D   ;
      )     ;
      =     "Gest DB Merker".App15;
NETWORK
TITLE =Asse B in Movimento verso il Secondo Posiz di Deposito Boxing DX
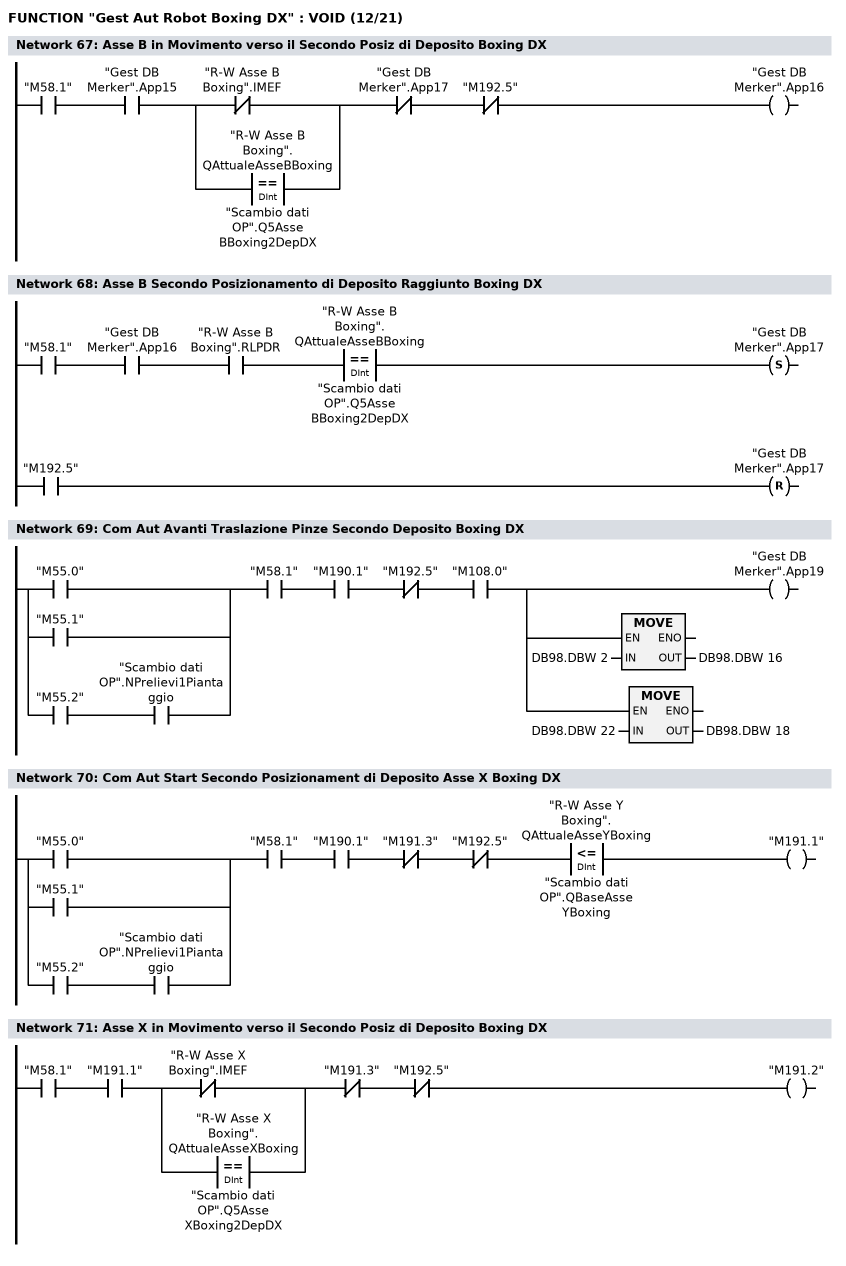
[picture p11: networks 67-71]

      U     "M58.1";
      U     "Gest DB Merker".App15;
      U(    ;
      ON    "R-W Asse B Boxing".IMEF;
      O(    ;
      L     "R-W Asse B Boxing".QAttualeAsseBBoxing;
      L     "Scambio dati OP".Q5AsseBBoxing2DepDX;
      ==D   ;
      )     ;
      )     ;
      UN    "Gest DB Merker".App17;
      UN    "M192.5";
      =     "Gest DB Merker".App16;
NETWORK
TITLE =Asse B Secondo Posizionamento di Deposito Raggiunto Boxing DX

      U     "M58.1";
      U     "Gest DB Merker".App16;
      U     "R-W Asse B Boxing".RLPDR;
      U(    ;
      L     "R-W Asse B Boxing".QAttualeAsseBBoxing;
      L     "Scambio dati OP".Q5AsseBBoxing2DepDX;
      ==D   ;
      )     ;
      S     "Gest DB Merker".App17;
      U     "M192.5";
      R     "Gest DB Merker".App17;
      NOP   0;
NETWORK
TITLE =Com Aut Avanti Traslazione Pinze Secondo Deposito Boxing DX

      U(    ;
      O     "M55.0";
      O     "M55.1";
      O     ;
      U     "M55.2";
      U     "Scambio dati OP".NPrelievi1Piantaggio;
      )     ;
      U     "M58.1";
      U     "M190.1";
      UN    "M192.5";
      U     "M108.0";
      =     L      0.0;
      U     L      0.0;
      BLD   102;
      =     "Gest DB Merker".App19;
      U     L      0.0;
      SPBNB _003;
      L     DB98.DBW    2;
      T     DB98.DBW   16;
_003: NOP   0;
      U     L      0.0;
      SPBNB _004;
      L     DB98.DBW   22;
      T     DB98.DBW   18;
_004: NOP   0;
NETWORK
TITLE =Com Aut Start Secondo Posizionament di Deposito Asse X Boxing DX

      U(    ;
      O     "M55.0";
      O     "M55.1";
      O     ;
      U     "M55.2";
      U     "Scambio dati OP".NPrelievi1Piantaggio;
      )     ;
      U     "M58.1";
      U     "M190.1";
      UN    "M191.3";
      UN    "M192.5";
      U(    ;
      L     "R-W Asse Y Boxing".QAttualeAsseYBoxing;
      L     "Scambio dati OP".QBaseAsseYBoxing;
      <=D   ;
      )     ;
      =     "M191.1";
NETWORK
TITLE =Asse X in Movimento verso il Secondo Posiz di Deposito Boxing DX

      U     "M58.1";
      U     "M191.1";
      U(    ;
      ON    "R-W Asse X Boxing".IMEF;
      O(    ;
      L     "R-W Asse X Boxing".QAttualeAsseXBoxing;
      L     "Scambio dati OP".Q5AsseXBoxing2DepDX;
      ==D   ;
      )     ;
      )     ;
      UN    "M191.3";
      UN    "M192.5";
      =     "M191.2";
NETWORK
TITLE =Asse X Secondo Posizionamento di Deposito Raggiunto Boxing DX
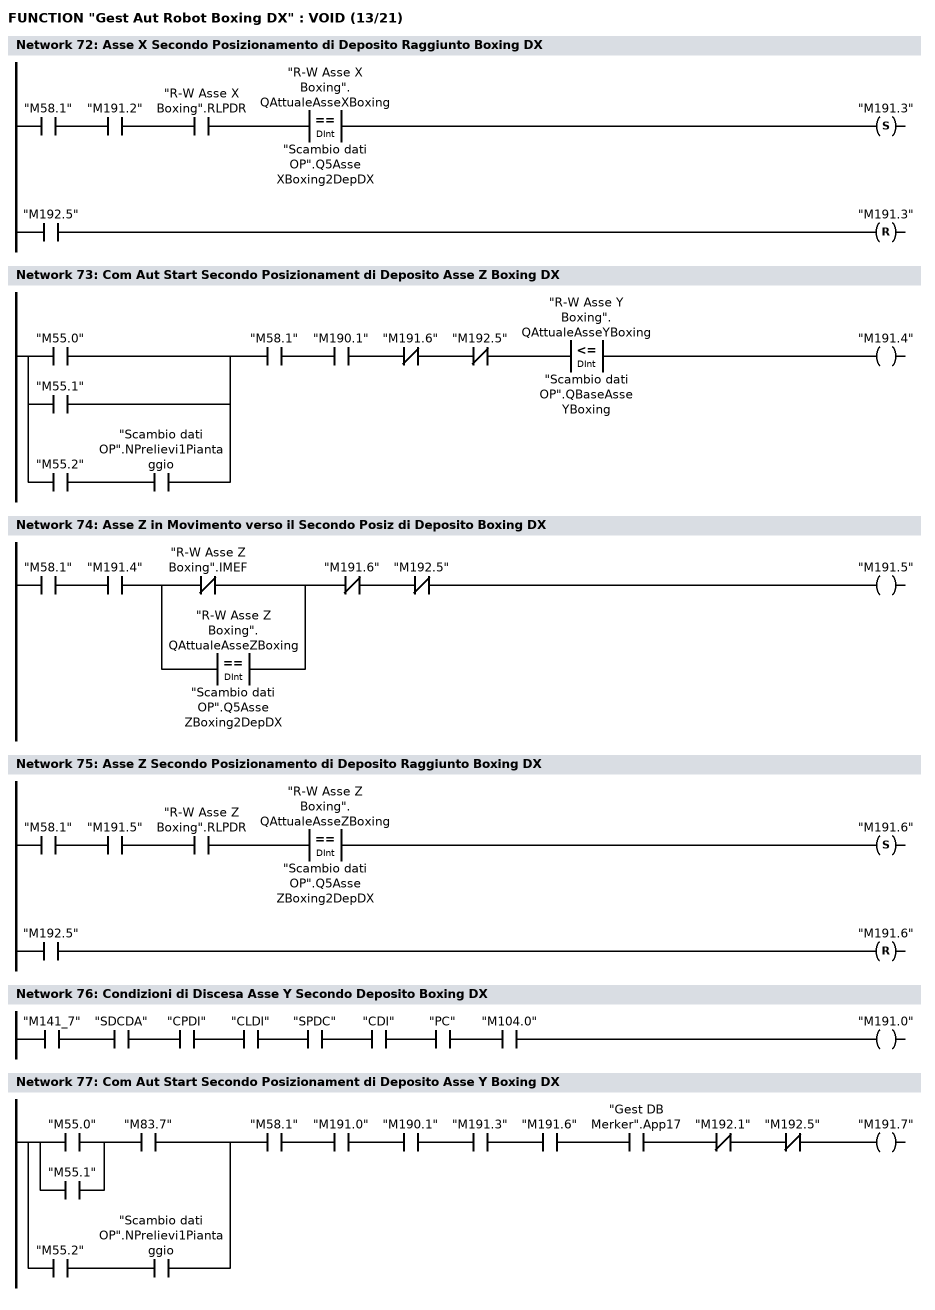
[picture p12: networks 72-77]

      U     "M58.1";
      U     "M191.2";
      U     "R-W Asse X Boxing".RLPDR;
      U(    ;
      L     "R-W Asse X Boxing".QAttualeAsseXBoxing;
      L     "Scambio dati OP".Q5AsseXBoxing2DepDX;
      ==D   ;
      )     ;
      S     "M191.3";
      U     "M192.5";
      R     "M191.3";
      NOP   0;
NETWORK
TITLE =Com Aut Start Secondo Posizionament di Deposito Asse Z Boxing DX

      U(    ;
      O     "M55.0";
      O     "M55.1";
      O     ;
      U     "M55.2";
      U     "Scambio dati OP".NPrelievi1Piantaggio;
      )     ;
      U     "M58.1";
      U     "M190.1";
      UN    "M191.6";
      UN    "M192.5";
      U(    ;
      L     "R-W Asse Y Boxing".QAttualeAsseYBoxing;
      L     "Scambio dati OP".QBaseAsseYBoxing;
      <=D   ;
      )     ;
      =     "M191.4";
NETWORK
TITLE =Asse Z in Movimento verso il Secondo Posiz di Deposito Boxing DX

      U     "M58.1";
      U     "M191.4";
      U(    ;
      ON    "R-W Asse Z Boxing".IMEF;
      O(    ;
      L     "R-W Asse Z Boxing".QAttualeAsseZBoxing;
      L     "Scambio dati OP".Q5AsseZBoxing2DepDX;
      ==D   ;
      )     ;
      )     ;
      UN    "M191.6";
      UN    "M192.5";
      =     "M191.5";
NETWORK
TITLE =Asse Z Secondo Posizionamento di Deposito Raggiunto Boxing DX

      U     "M58.1";
      U     "M191.5";
      U     "R-W Asse Z Boxing".RLPDR;
      U(    ;
      L     "R-W Asse Z Boxing".QAttualeAsseZBoxing;
      L     "Scambio dati OP".Q5AsseZBoxing2DepDX;
      ==D   ;
      )     ;
      S     "M191.6";
      U     "M192.5";
      R     "M191.6";
      NOP   0;
NETWORK
TITLE =Condizioni di Discesa Asse Y Secondo Deposito Boxing DX

      U     "M141_7";
      U     "SDCDA";
      U     "CPDI";
      U     "CLDI";
      U     "SPDC";
      U     "CDI";
      U     "PC";
      U     "M104.0";
      =     "M191.0";
NETWORK
TITLE =Com Aut Start Secondo Posizionament di Deposito Asse Y Boxing DX

      U(    ;
      U(    ;
      O     "M55.0";
      O     "M55.1";
      )     ;
      U     "M83.7";
      O     ;
      U     "M55.2";
      U     "Scambio dati OP".NPrelievi1Piantaggio;
      )     ;
      U     "M58.1";
      U     "M191.0";
      U     "M190.1";
      U     "M191.3";
      U     "M191.6";
      U     "Gest DB Merker".App17;
      UN    "M192.1";
      UN    "M192.5";
      =     "M191.7";
NETWORK
TITLE =Asse Y in Moviment verso il Secondo Posiz di Deposito Boxing DX
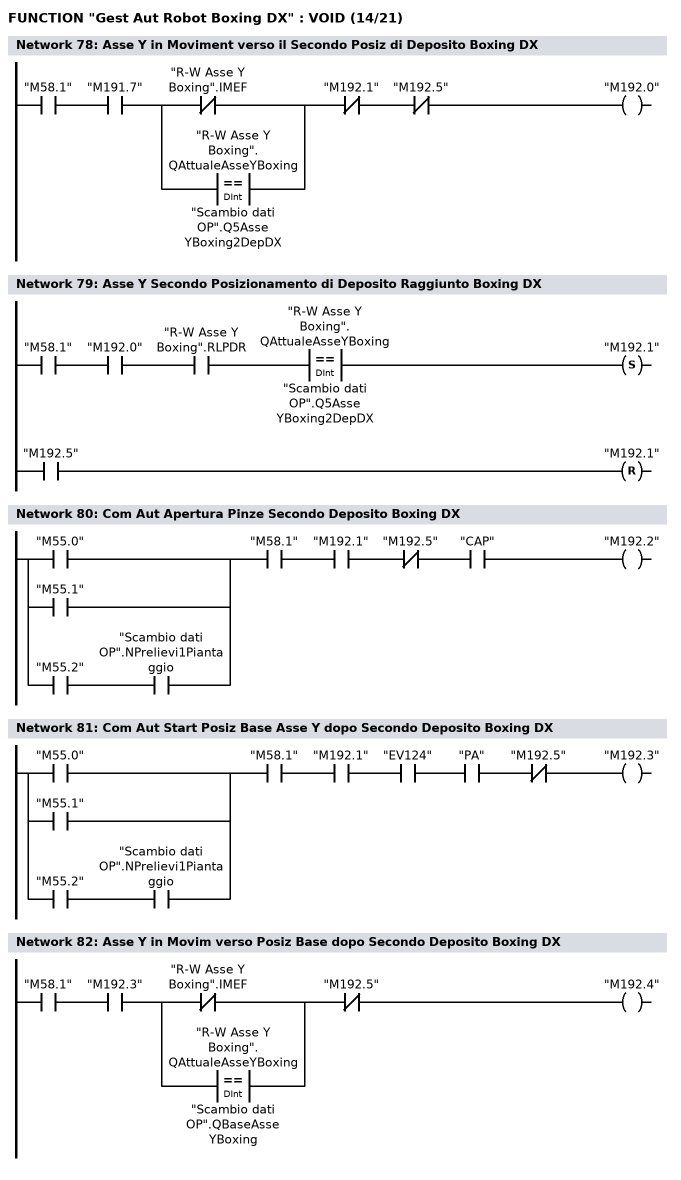
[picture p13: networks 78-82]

      U     "M58.1";
      U     "M191.7";
      U(    ;
      ON    "R-W Asse Y Boxing".IMEF;
      O(    ;
      L     "R-W Asse Y Boxing".QAttualeAsseYBoxing;
      L     "Scambio dati OP".Q5AsseYBoxing2DepDX;
      ==D   ;
      )     ;
      )     ;
      UN    "M192.1";
      UN    "M192.5";
      =     "M192.0";
NETWORK
TITLE =Asse Y Secondo Posizionamento di Deposito Raggiunto Boxing DX

      U     "M58.1";
      U     "M192.0";
      U     "R-W Asse Y Boxing".RLPDR;
      U(    ;
      L     "R-W Asse Y Boxing".QAttualeAsseYBoxing;
      L     "Scambio dati OP".Q5AsseYBoxing2DepDX;
      ==D   ;
      )     ;
      S     "M192.1";
      U     "M192.5";
      R     "M192.1";
      NOP   0;
NETWORK
TITLE =Com Aut Apertura Pinze Secondo Deposito Boxing DX

      U(    ;
      O     "M55.0";
      O     "M55.1";
      O     ;
      U     "M55.2";
      U     "Scambio dati OP".NPrelievi1Piantaggio;
      )     ;
      U     "M58.1";
      U     "M192.1";
      UN    "M192.5";
      U     "CAP";
      =     "M192.2";
NETWORK
TITLE =Com Aut Start Posiz Base Asse Y dopo Secondo Deposito Boxing DX

      U(    ;
      O     "M55.0";
      O     "M55.1";
      O     ;
      U     "M55.2";
      U     "Scambio dati OP".NPrelievi1Piantaggio;
      )     ;
      U     "M58.1";
      U     "M192.1";
      U     "EV124";
      U     "PA";
      UN    "M192.5";
      =     "M192.3";
NETWORK
TITLE =Asse Y in Movim verso Posiz Base dopo Secondo Deposito Boxing DX

      U     "M58.1";
      U     "M192.3";
      U(    ;
      ON    "R-W Asse Y Boxing".IMEF;
      O(    ;
      L     "R-W Asse Y Boxing".QAttualeAsseYBoxing;
      L     "Scambio dati OP".QBaseAsseYBoxing;
      ==D   ;
      )     ;
      )     ;
      UN    "M192.5";
      =     "M192.4";
NETWORK
TITLE =Asse Y Posizione Base dopo Secondo Deposito Raggiunta Boxing DX
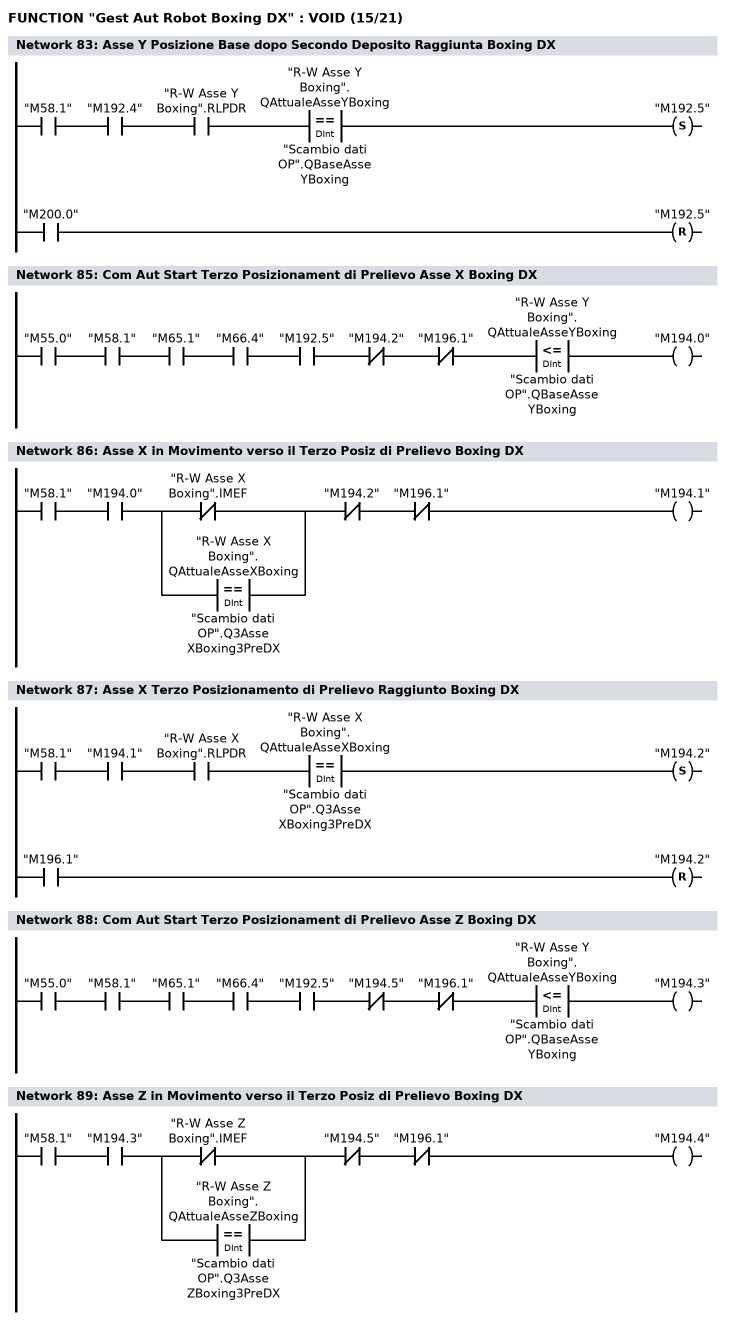
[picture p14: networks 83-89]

      U     "M58.1";
      U     "M192.4";
      U     "R-W Asse Y Boxing".RLPDR;
      U(    ;
      L     "R-W Asse Y Boxing".QAttualeAsseYBoxing;
      L     "Scambio dati OP".QBaseAsseYBoxing;
      ==D   ;
      )     ;
      S     "M192.5";
      U     "M200.0";
      R     "M192.5";
      NOP   0;
NETWORK
TITLE ======== Terzo Prelievo Ciclo 3 Pinataggi Boxing =======



NETWORK
TITLE =Com Aut Start Terzo Posizionament di Prelievo Asse X Boxing DX

      U     "M55.0";
      U     "M58.1";
      U     "M65.1";
      U     "M66.4";
      U     "M192.5";
      UN    "M194.2";
      UN    "M196.1";
      U(    ;
      L     "R-W Asse Y Boxing".QAttualeAsseYBoxing;
      L     "Scambio dati OP".QBaseAsseYBoxing;
      <=D   ;
      )     ;
      =     "M194.0";
NETWORK
TITLE =Asse X in Movimento verso il Terzo Posiz di Prelievo Boxing DX

      U     "M58.1";
      U     "M194.0";
      U(    ;
      ON    "R-W Asse X Boxing".IMEF;
      O(    ;
      L     "R-W Asse X Boxing".QAttualeAsseXBoxing;
      L     "Scambio dati OP".Q3AsseXBoxing3PreDX;
      ==D   ;
      )     ;
      )     ;
      UN    "M194.2";
      UN    "M196.1";
      =     "M194.1";
NETWORK
TITLE =Asse X Terzo Posizionamento di Prelievo Raggiunto Boxing DX

      U     "M58.1";
      U     "M194.1";
      U     "R-W Asse X Boxing".RLPDR;
      U(    ;
      L     "R-W Asse X Boxing".QAttualeAsseXBoxing;
      L     "Scambio dati OP".Q3AsseXBoxing3PreDX;
      ==D   ;
      )     ;
      S     "M194.2";
      U     "M196.1";
      R     "M194.2";
      NOP   0;
NETWORK
TITLE =Com Aut Start Terzo Posizionament di Prelievo Asse Z Boxing DX

      U     "M55.0";
      U     "M58.1";
      U     "M65.1";
      U     "M66.4";
      U     "M192.5";
      UN    "M194.5";
      UN    "M196.1";
      U(    ;
      L     "R-W Asse Y Boxing".QAttualeAsseYBoxing;
      L     "Scambio dati OP".QBaseAsseYBoxing;
      <=D   ;
      )     ;
      =     "M194.3";
NETWORK
TITLE =Asse Z in Movimento verso il Terzo Posiz di Prelievo Boxing DX

      U     "M58.1";
      U     "M194.3";
      U(    ;
      ON    "R-W Asse Z Boxing".IMEF;
      O(    ;
      L     "R-W Asse Z Boxing".QAttualeAsseZBoxing;
      L     "Scambio dati OP".Q3AsseZBoxing3PreDX;
      ==D   ;
      )     ;
      )     ;
      UN    "M194.5";
      UN    "M196.1";
      =     "M194.4";
NETWORK
TITLE =Asse Z Terzo Posizionamento di Prelievo Raggiunto Boxing DX
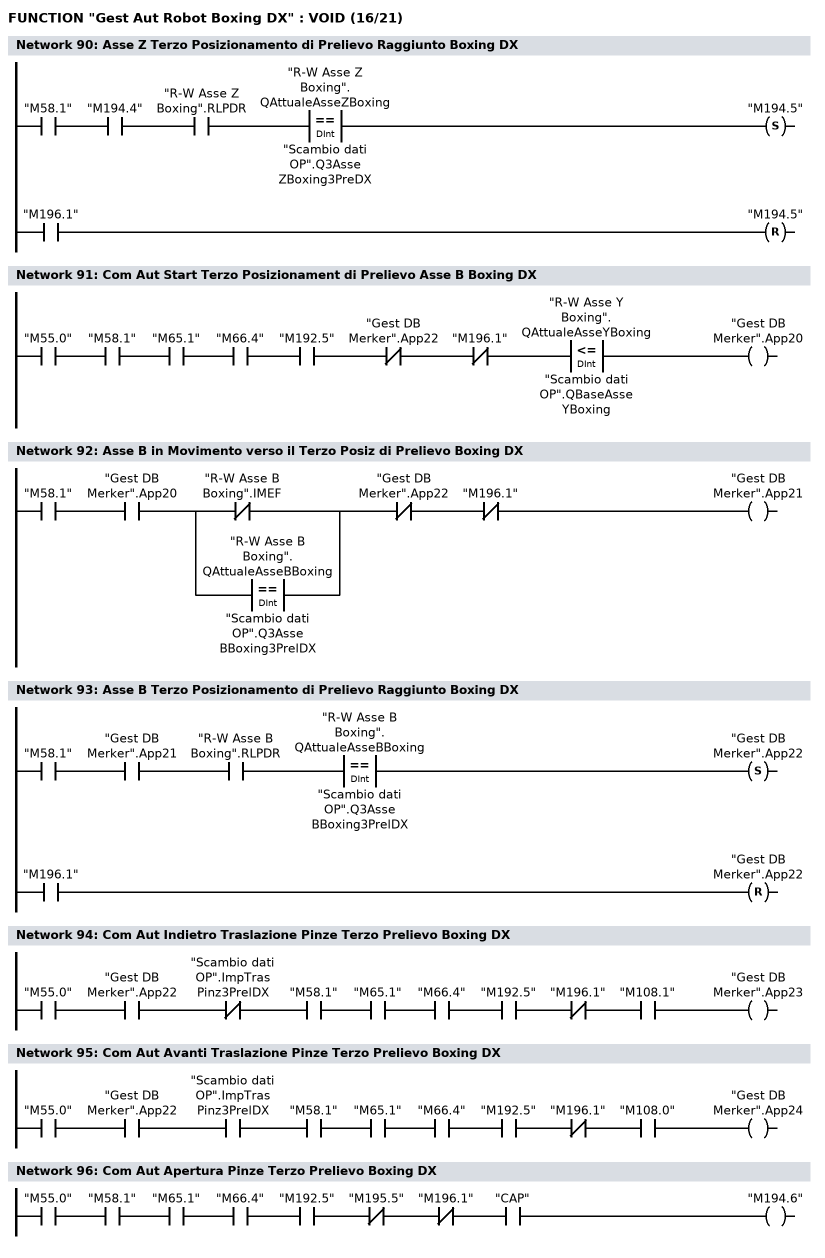
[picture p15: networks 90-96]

      U     "M58.1";
      U     "M194.4";
      U     "R-W Asse Z Boxing".RLPDR;
      U(    ;
      L     "R-W Asse Z Boxing".QAttualeAsseZBoxing;
      L     "Scambio dati OP".Q3AsseZBoxing3PreDX;
      ==D   ;
      )     ;
      S     "M194.5";
      U     "M196.1";
      R     "M194.5";
      NOP   0;
NETWORK
TITLE =Com Aut Start Terzo Posizionament di Prelievo Asse B Boxing DX

      U     "M55.0";
      U     "M58.1";
      U     "M65.1";
      U     "M66.4";
      U     "M192.5";
      UN    "Gest DB Merker".App22;
      UN    "M196.1";
      U(    ;
      L     "R-W Asse Y Boxing".QAttualeAsseYBoxing;
      L     "Scambio dati OP".QBaseAsseYBoxing;
      <=D   ;
      )     ;
      =     "Gest DB Merker".App20;
NETWORK
TITLE =Asse B in Movimento verso il Terzo Posiz di Prelievo Boxing DX

      U     "M58.1";
      U     "Gest DB Merker".App20;
      U(    ;
      ON    "R-W Asse B Boxing".IMEF;
      O(    ;
      L     "R-W Asse B Boxing".QAttualeAsseBBoxing;
      L     "Scambio dati OP".Q3AsseBBoxing3PrelDX;
      ==D   ;
      )     ;
      )     ;
      UN    "Gest DB Merker".App22;
      UN    "M196.1";
      =     "Gest DB Merker".App21;
NETWORK
TITLE =Asse B Terzo Posizionamento di Prelievo Raggiunto Boxing DX

      U     "M58.1";
      U     "Gest DB Merker".App21;
      U     "R-W Asse B Boxing".RLPDR;
      U(    ;
      L     "R-W Asse B Boxing".QAttualeAsseBBoxing;
      L     "Scambio dati OP".Q3AsseBBoxing3PrelDX;
      ==D   ;
      )     ;
      S     "Gest DB Merker".App22;
      U     "M196.1";
      R     "Gest DB Merker".App22;
      NOP   0;
NETWORK
TITLE =Com Aut Indietro Traslazione Pinze Terzo Prelievo Boxing DX

      U     "M55.0";
      U     "Gest DB Merker".App22;
      UN    "Scambio dati OP".ImpTrasPinz3PrelDX;
      U     "M58.1";
      U     "M65.1";
      U     "M66.4";
      U     "M192.5";
      UN    "M196.1";
      U     "M108.1";
      =     "Gest DB Merker".App23;
NETWORK
TITLE =Com Aut Avanti Traslazione Pinze Terzo Prelievo Boxing DX

      U     "M55.0";
      U     "Gest DB Merker".App22;
      U     "Scambio dati OP".ImpTrasPinz3PrelDX;
      U     "M58.1";
      U     "M65.1";
      U     "M66.4";
      U     "M192.5";
      UN    "M196.1";
      U     "M108.0";
      =     "Gest DB Merker".App24;
NETWORK
TITLE =Com Aut Apertura Pinze Terzo Prelievo Boxing DX

      U     "M55.0";
      U     "M58.1";
      U     "M65.1";
      U     "M66.4";
      U     "M192.5";
      UN    "M195.5";
      UN    "M196.1";
      U     "CAP";
      =     "M194.6";
NETWORK
TITLE =Condizioni di Discesa Asse Y Terzo Prelievo Boxing DX
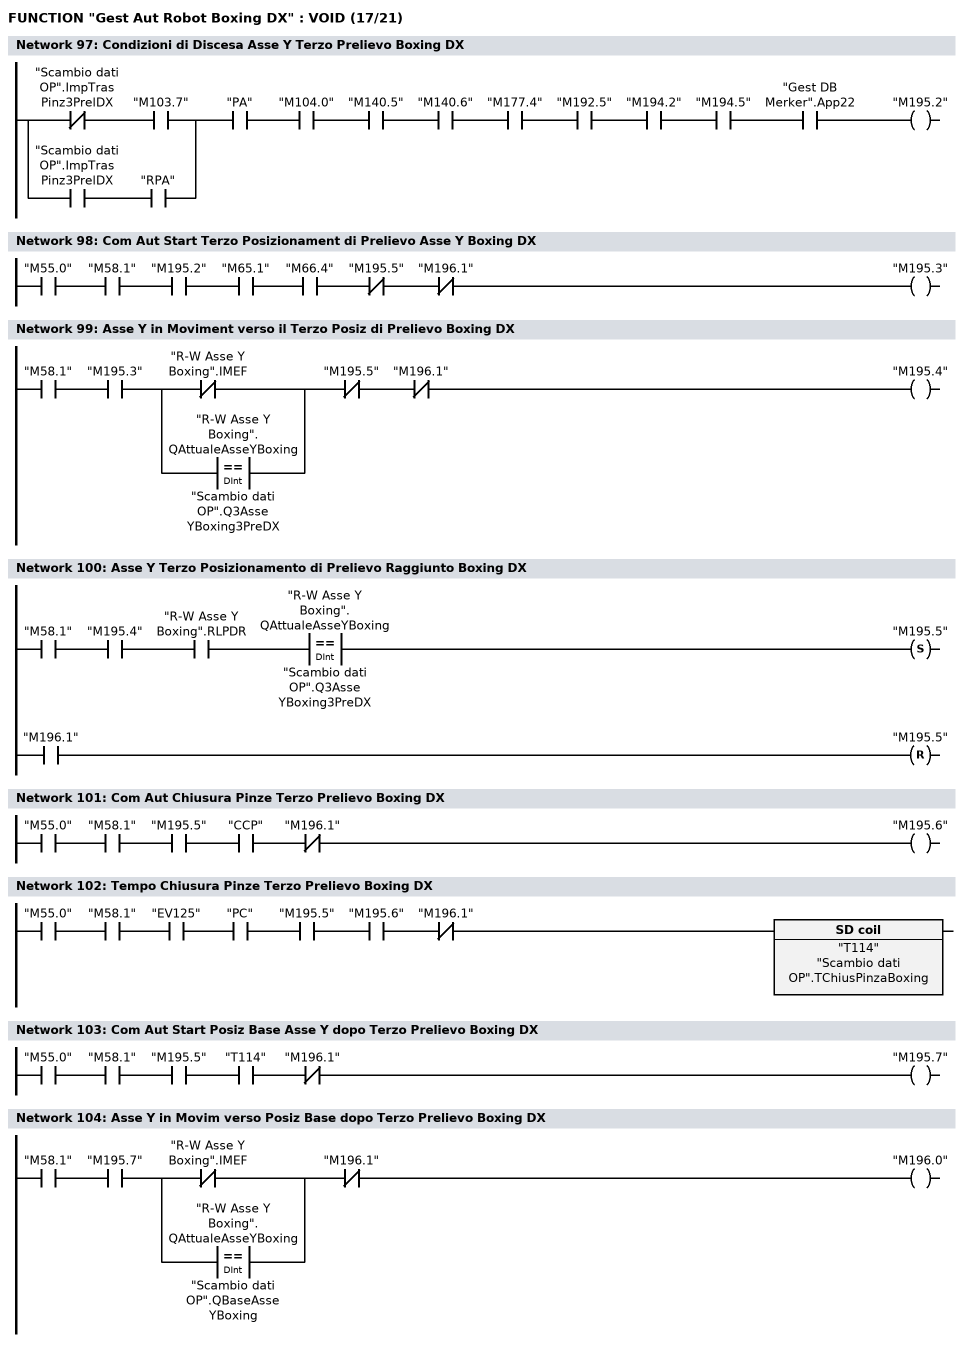
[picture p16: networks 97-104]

      U(    ;
      UN    "Scambio dati OP".ImpTrasPinz3PrelDX;
      U     "M103.7";
      O     ;
      U     "Scambio dati OP".ImpTrasPinz3PrelDX;
      U     "RPA";
      )     ;
      U     "PA";
      U     "M104.0";
      U     "M140.5";
      U     "M140.6";
      U     "M177.4";
      U     "M192.5";
      U     "M194.2";
      U     "M194.5";
      U     "Gest DB Merker".App22;
      =     "M195.2";
NETWORK
TITLE =Com Aut Start Terzo Posizionament di Prelievo Asse Y Boxing DX

      U     "M55.0";
      U     "M58.1";
      U     "M195.2";
      U     "M65.1";
      U     "M66.4";
      UN    "M195.5";
      UN    "M196.1";
      =     "M195.3";
NETWORK
TITLE =Asse Y in Moviment verso il Terzo Posiz di Prelievo Boxing DX

      U     "M58.1";
      U     "M195.3";
      U(    ;
      ON    "R-W Asse Y Boxing".IMEF;
      O(    ;
      L     "R-W Asse Y Boxing".QAttualeAsseYBoxing;
      L     "Scambio dati OP".Q3AsseYBoxing3PreDX;
      ==D   ;
      )     ;
      )     ;
      UN    "M195.5";
      UN    "M196.1";
      =     "M195.4";
NETWORK
TITLE =Asse Y Terzo Posizionamento di Prelievo Raggiunto Boxing DX

      U     "M58.1";
      U     "M195.4";
      U     "R-W Asse Y Boxing".RLPDR;
      U(    ;
      L     "R-W Asse Y Boxing".QAttualeAsseYBoxing;
      L     "Scambio dati OP".Q3AsseYBoxing3PreDX;
      ==D   ;
      )     ;
      S     "M195.5";
      U     "M196.1";
      R     "M195.5";
      NOP   0;
NETWORK
TITLE =Com Aut Chiusura Pinze Terzo Prelievo Boxing DX

      U     "M55.0";
      U     "M58.1";
      U     "M195.5";
      U     "CCP";
      UN    "M196.1";
      =     "M195.6";
NETWORK
TITLE =Tempo Chiusura Pinze Terzo Prelievo Boxing DX

      U     "M55.0";
      U     "M58.1";
      U     "EV125";
      U     "PC";
      U     "M195.5";
      U     "M195.6";
      UN    "M196.1";
      L     "Scambio dati OP".TChiusPinzaBoxing;
      SE    "T114";
      NOP   0;
      NOP   0;
      NOP   0;
      NOP   0;
NETWORK
TITLE =Com Aut Start Posiz Base Asse Y dopo Terzo Prelievo Boxing DX

      U     "M55.0";
      U     "M58.1";
      U     "M195.5";
      U     "T114";
      UN    "M196.1";
      =     "M195.7";
NETWORK
TITLE =Asse Y in Movim verso Posiz Base dopo Terzo Prelievo Boxing DX

      U     "M58.1";
      U     "M195.7";
      U(    ;
      ON    "R-W Asse Y Boxing".IMEF;
      O(    ;
      L     "R-W Asse Y Boxing".QAttualeAsseYBoxing;
      L     "Scambio dati OP".QBaseAsseYBoxing;
      ==D   ;
      )     ;
      )     ;
      UN    "M196.1";
      =     "M196.0";
NETWORK
TITLE =Asse Y Posizione Base dopo Terzo Prelievo Raggiunta Boxing DX
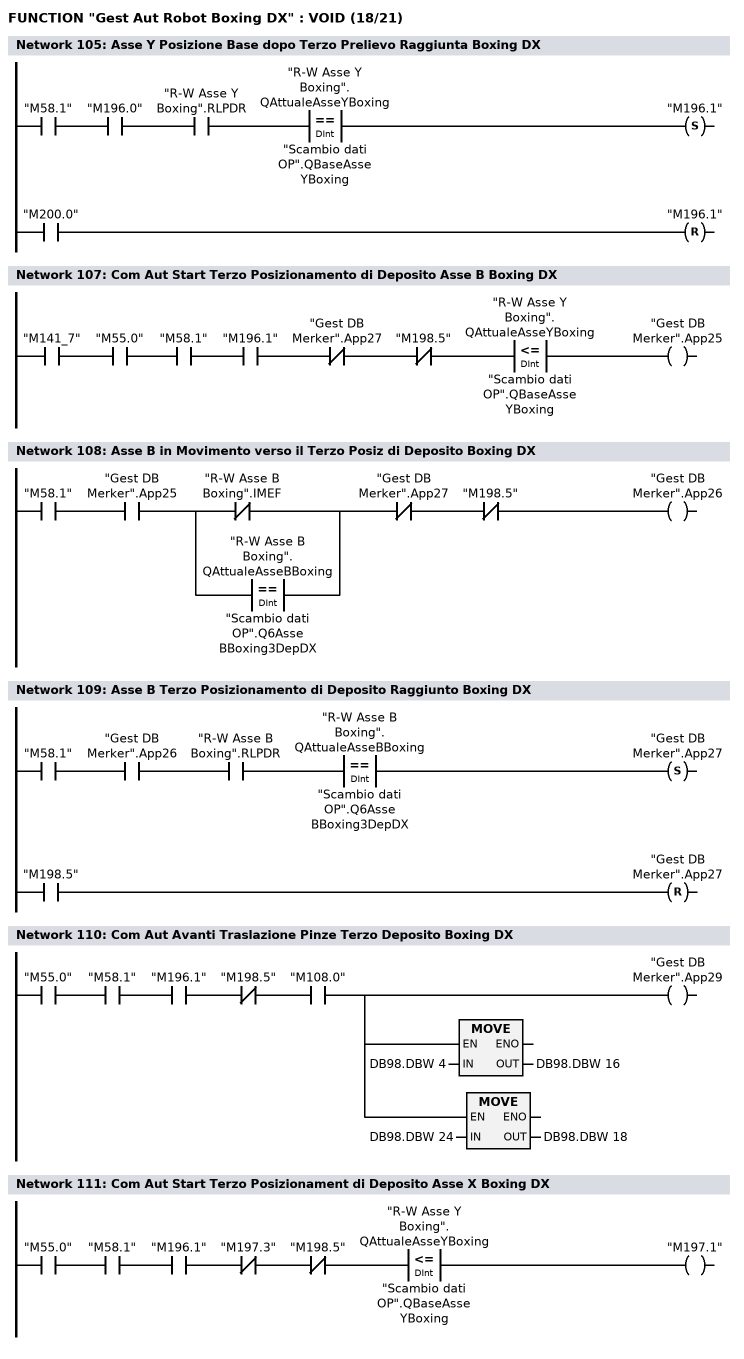
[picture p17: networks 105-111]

      U     "M58.1";
      U     "M196.0";
      U     "R-W Asse Y Boxing".RLPDR;
      U(    ;
      L     "R-W Asse Y Boxing".QAttualeAsseYBoxing;
      L     "Scambio dati OP".QBaseAsseYBoxing;
      ==D   ;
      )     ;
      S     "M196.1";
      U     "M200.0";
      R     "M196.1";
      NOP   0;
NETWORK
TITLE ======== Terzo Deposito Ciclo 3 Pinataggi Boxing =======



NETWORK
TITLE =Com Aut Start Terzo Posizionamento di Deposito Asse B Boxing DX

      U     "M141_7";
      U     "M55.0";
      U     "M58.1";
      U     "M196.1";
      UN    "Gest DB Merker".App27;
      UN    "M198.5";
      U(    ;
      L     "R-W Asse Y Boxing".QAttualeAsseYBoxing;
      L     "Scambio dati OP".QBaseAsseYBoxing;
      <=D   ;
      )     ;
      =     "Gest DB Merker".App25;
NETWORK
TITLE =Asse B in Movimento verso il Terzo Posiz di Deposito Boxing DX

      U     "M58.1";
      U     "Gest DB Merker".App25;
      U(    ;
      ON    "R-W Asse B Boxing".IMEF;
      O(    ;
      L     "R-W Asse B Boxing".QAttualeAsseBBoxing;
      L     "Scambio dati OP".Q6AsseBBoxing3DepDX;
      ==D   ;
      )     ;
      )     ;
      UN    "Gest DB Merker".App27;
      UN    "M198.5";
      =     "Gest DB Merker".App26;
NETWORK
TITLE =Asse B Terzo Posizionamento di Deposito Raggiunto Boxing DX

      U     "M58.1";
      U     "Gest DB Merker".App26;
      U     "R-W Asse B Boxing".RLPDR;
      U(    ;
      L     "R-W Asse B Boxing".QAttualeAsseBBoxing;
      L     "Scambio dati OP".Q6AsseBBoxing3DepDX;
      ==D   ;
      )     ;
      S     "Gest DB Merker".App27;
      U     "M198.5";
      R     "Gest DB Merker".App27;
      NOP   0;
NETWORK
TITLE =Com Aut Avanti Traslazione Pinze Terzo Deposito Boxing DX

      U     "M55.0";
      U     "M58.1";
      U     "M196.1";
      UN    "M198.5";
      U     "M108.0";
      =     L      0.0;
      U     L      0.0;
      BLD   102;
      =     "Gest DB Merker".App29;
      U     L      0.0;
      SPBNB _005;
      L     DB98.DBW    4;
      T     DB98.DBW   16;
_005: NOP   0;
      U     L      0.0;
      SPBNB _006;
      L     DB98.DBW   24;
      T     DB98.DBW   18;
_006: NOP   0;
NETWORK
TITLE =Com Aut Start Terzo Posizionament di Deposito Asse X Boxing DX

      U     "M55.0";
      U     "M58.1";
      U     "M196.1";
      UN    "M197.3";
      UN    "M198.5";
      U(    ;
      L     "R-W Asse Y Boxing".QAttualeAsseYBoxing;
      L     "Scambio dati OP".QBaseAsseYBoxing;
      <=D   ;
      )     ;
      =     "M197.1";
NETWORK
TITLE =Asse X in Movimento verso il Terzo Posiz di Deposito Boxing DX
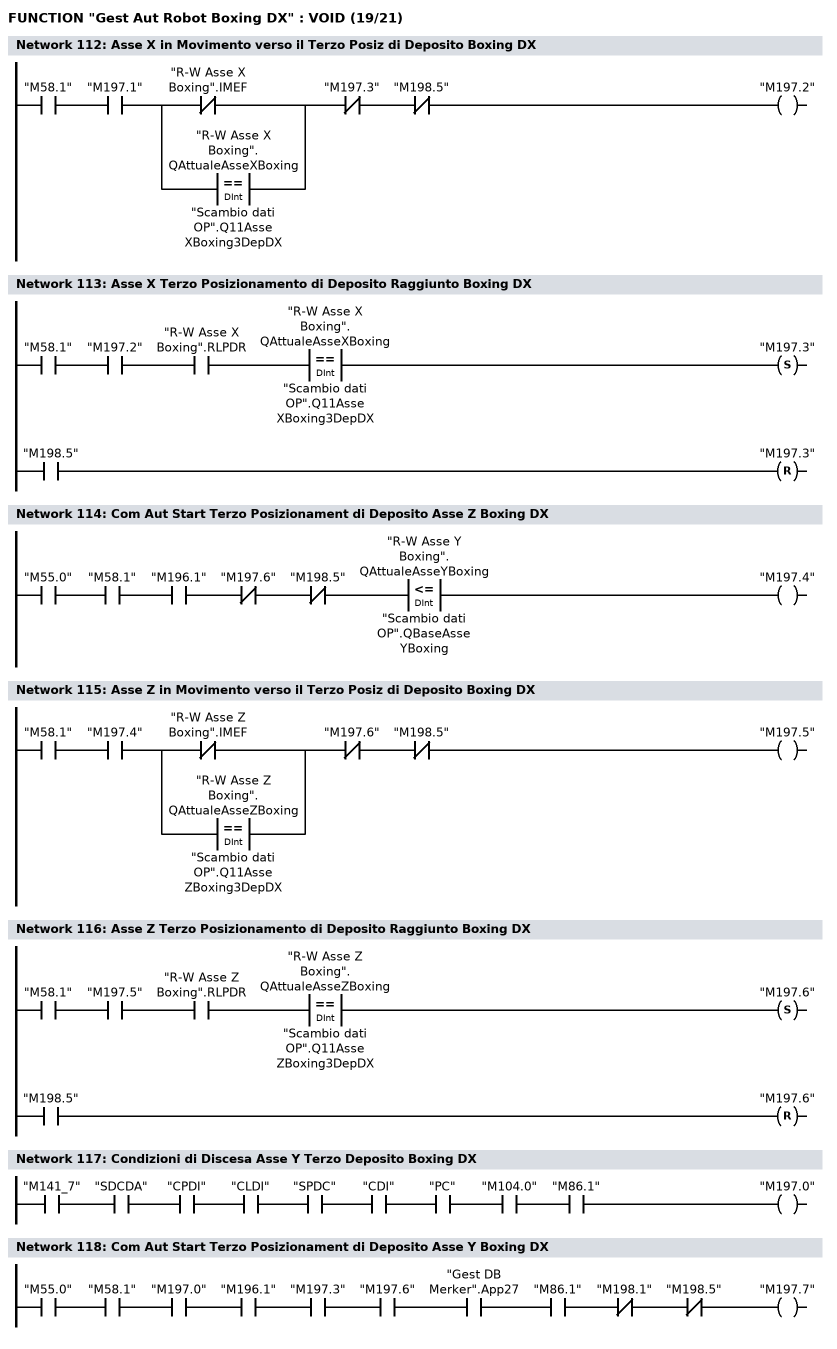
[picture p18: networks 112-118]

      U     "M58.1";
      U     "M197.1";
      U(    ;
      ON    "R-W Asse X Boxing".IMEF;
      O(    ;
      L     "R-W Asse X Boxing".QAttualeAsseXBoxing;
      L     "Scambio dati OP".Q11AsseXBoxing3DepDX;
      ==D   ;
      )     ;
      )     ;
      UN    "M197.3";
      UN    "M198.5";
      =     "M197.2";
NETWORK
TITLE =Asse X Terzo Posizionamento di Deposito Raggiunto Boxing DX

      U     "M58.1";
      U     "M197.2";
      U     "R-W Asse X Boxing".RLPDR;
      U(    ;
      L     "R-W Asse X Boxing".QAttualeAsseXBoxing;
      L     "Scambio dati OP".Q11AsseXBoxing3DepDX;
      ==D   ;
      )     ;
      S     "M197.3";
      U     "M198.5";
      R     "M197.3";
      NOP   0;
NETWORK
TITLE =Com Aut Start Terzo Posizionament di Deposito Asse Z Boxing DX

      U     "M55.0";
      U     "M58.1";
      U     "M196.1";
      UN    "M197.6";
      UN    "M198.5";
      U(    ;
      L     "R-W Asse Y Boxing".QAttualeAsseYBoxing;
      L     "Scambio dati OP".QBaseAsseYBoxing;
      <=D   ;
      )     ;
      =     "M197.4";
NETWORK
TITLE =Asse Z in Movimento verso il Terzo Posiz di Deposito Boxing DX

      U     "M58.1";
      U     "M197.4";
      U(    ;
      ON    "R-W Asse Z Boxing".IMEF;
      O(    ;
      L     "R-W Asse Z Boxing".QAttualeAsseZBoxing;
      L     "Scambio dati OP".Q11AsseZBoxing3DepDX;
      ==D   ;
      )     ;
      )     ;
      UN    "M197.6";
      UN    "M198.5";
      =     "M197.5";
NETWORK
TITLE =Asse Z Terzo Posizionamento di Deposito Raggiunto Boxing DX

      U     "M58.1";
      U     "M197.5";
      U     "R-W Asse Z Boxing".RLPDR;
      U(    ;
      L     "R-W Asse Z Boxing".QAttualeAsseZBoxing;
      L     "Scambio dati OP".Q11AsseZBoxing3DepDX;
      ==D   ;
      )     ;
      S     "M197.6";
      U     "M198.5";
      R     "M197.6";
      NOP   0;
NETWORK
TITLE =Condizioni di Discesa Asse Y Terzo Deposito Boxing DX

      U     "M141_7";
      U     "SDCDA";
      U     "CPDI";
      U     "CLDI";
      U     "SPDC";
      U     "CDI";
      U     "PC";
      U     "M104.0";
      U     "M86.1";
      =     "M197.0";
NETWORK
TITLE =Com Aut Start Terzo Posizionament di Deposito Asse Y Boxing DX

      U     "M55.0";
      U     "M58.1";
      U     "M197.0";
      U     "M196.1";
      U     "M197.3";
      U     "M197.6";
      U     "Gest DB Merker".App27;
      U     "M86.1";
      UN    "M198.1";
      UN    "M198.5";
      =     "M197.7";
NETWORK
TITLE =Asse Y in Moviment verso il Terzo Posiz di Deposito Boxing DX
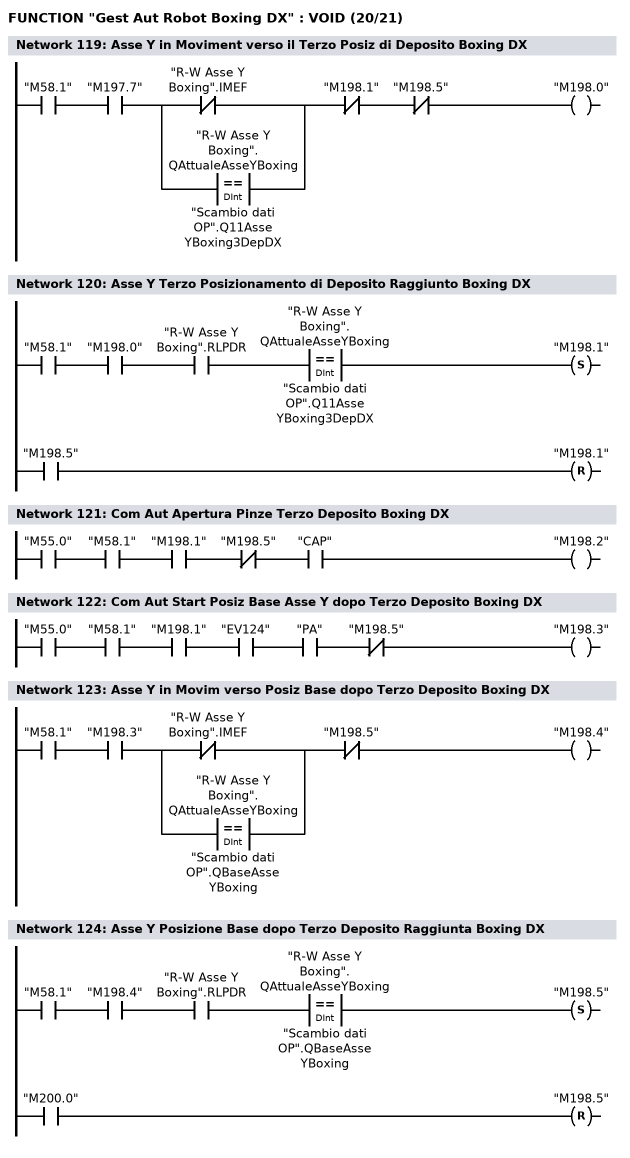
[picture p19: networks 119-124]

      U     "M58.1";
      U     "M197.7";
      U(    ;
      ON    "R-W Asse Y Boxing".IMEF;
      O(    ;
      L     "R-W Asse Y Boxing".QAttualeAsseYBoxing;
      L     "Scambio dati OP".Q11AsseYBoxing3DepDX;
      ==D   ;
      )     ;
      )     ;
      UN    "M198.1";
      UN    "M198.5";
      =     "M198.0";
NETWORK
TITLE =Asse Y Terzo Posizionamento di Deposito Raggiunto Boxing DX

      U     "M58.1";
      U     "M198.0";
      U     "R-W Asse Y Boxing".RLPDR;
      U(    ;
      L     "R-W Asse Y Boxing".QAttualeAsseYBoxing;
      L     "Scambio dati OP".Q11AsseYBoxing3DepDX;
      ==D   ;
      )     ;
      S     "M198.1";
      U     "M198.5";
      R     "M198.1";
      NOP   0;
NETWORK
TITLE =Com Aut Apertura Pinze Terzo Deposito Boxing DX

      U     "M55.0";
      U     "M58.1";
      U     "M198.1";
      UN    "M198.5";
      U     "CAP";
      =     "M198.2";
NETWORK
TITLE =Com Aut Start Posiz Base Asse Y dopo Terzo Deposito Boxing DX

      U     "M55.0";
      U     "M58.1";
      U     "M198.1";
      U     "EV124";
      U     "PA";
      UN    "M198.5";
      =     "M198.3";
NETWORK
TITLE =Asse Y in Movim verso Posiz Base dopo Terzo Deposito Boxing DX

      U     "M58.1";
      U     "M198.3";
      U(    ;
      ON    "R-W Asse Y Boxing".IMEF;
      O(    ;
      L     "R-W Asse Y Boxing".QAttualeAsseYBoxing;
      L     "Scambio dati OP".QBaseAsseYBoxing;
      ==D   ;
      )     ;
      )     ;
      UN    "M198.5";
      =     "M198.4";
NETWORK
TITLE =Asse Y Posizione Base dopo Terzo Deposito Raggiunta Boxing DX

      U     "M58.1";
      U     "M198.4";
      U     "R-W Asse Y Boxing".RLPDR;
      U(    ;
      L     "R-W Asse Y Boxing".QAttualeAsseYBoxing;
      L     "Scambio dati OP".QBaseAsseYBoxing;
      ==D   ;
      )     ;
      S     "M198.5";
      U     "M200.0";
      R     "M198.5";
      NOP   0;
NETWORK
TITLE =Fine Ciclo Totale Boxing DX
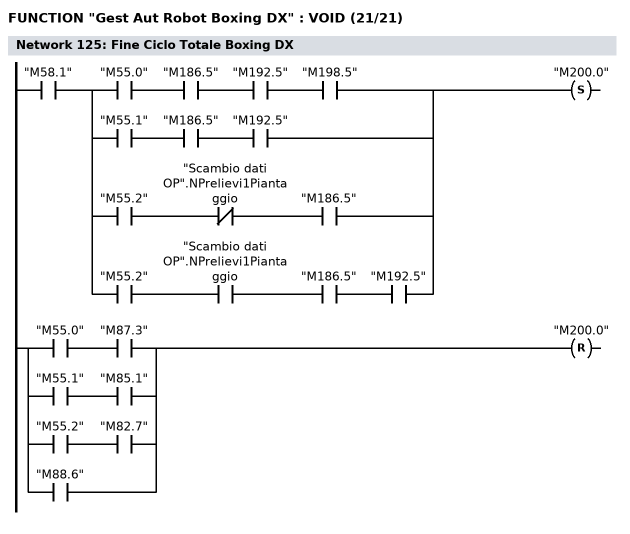
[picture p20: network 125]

      U     "M58.1";
      U(    ;
      U     "M55.0";
      U     "M186.5";
      U     "M192.5";
      U     "M198.5";
      O     ;
      U     "M55.1";
      U     "M186.5";
      U     "M192.5";
      O     ;
      U     "M55.2";
      UN    "Scambio dati OP".NPrelievi1Piantaggio;
      U     "M186.5";
      O     ;
      U     "M55.2";
      U     "Scambio dati OP".NPrelievi1Piantaggio;
      U     "M186.5";
      U     "M192.5";
      )     ;
      S     "M200.0";
      U(    ;
      U     "M55.0";
      U     "M87.3";
      O     ;
      U     "M55.1";
      U     "M85.1";
      O     ;
      U     "M55.2";
      U     "M82.7";
      O     "M88.6";
      )     ;
      R     "M200.0";
      NOP   0;
END_FUNCTION

